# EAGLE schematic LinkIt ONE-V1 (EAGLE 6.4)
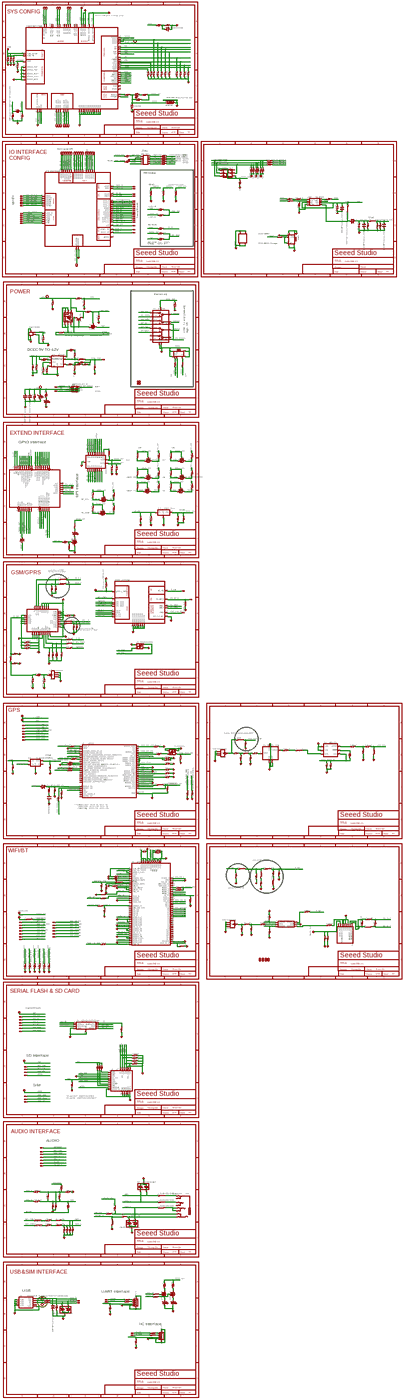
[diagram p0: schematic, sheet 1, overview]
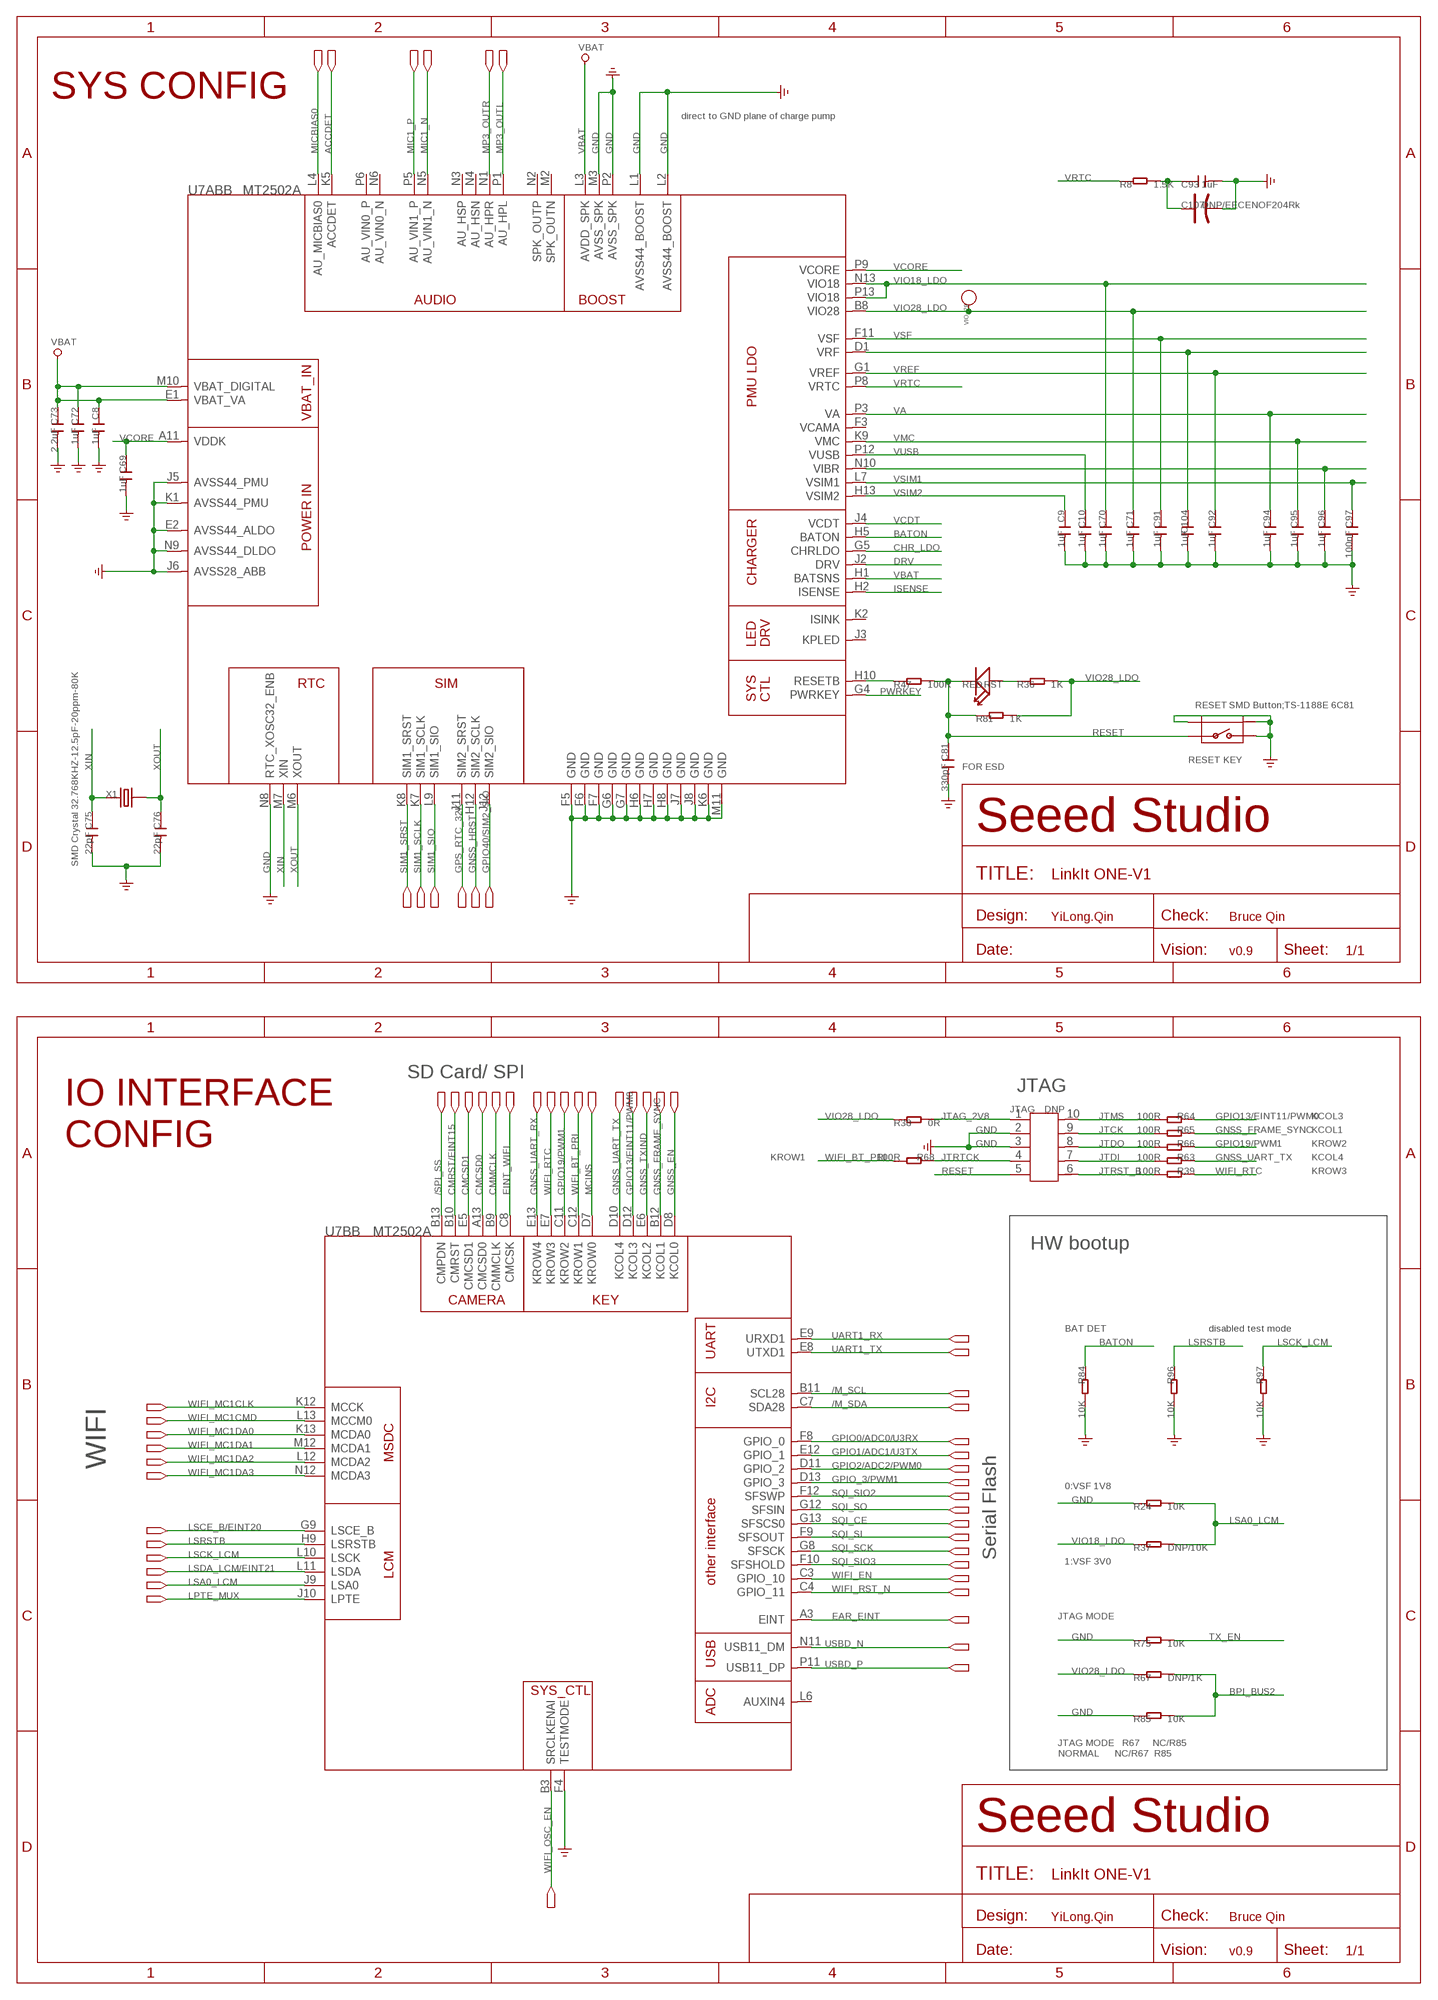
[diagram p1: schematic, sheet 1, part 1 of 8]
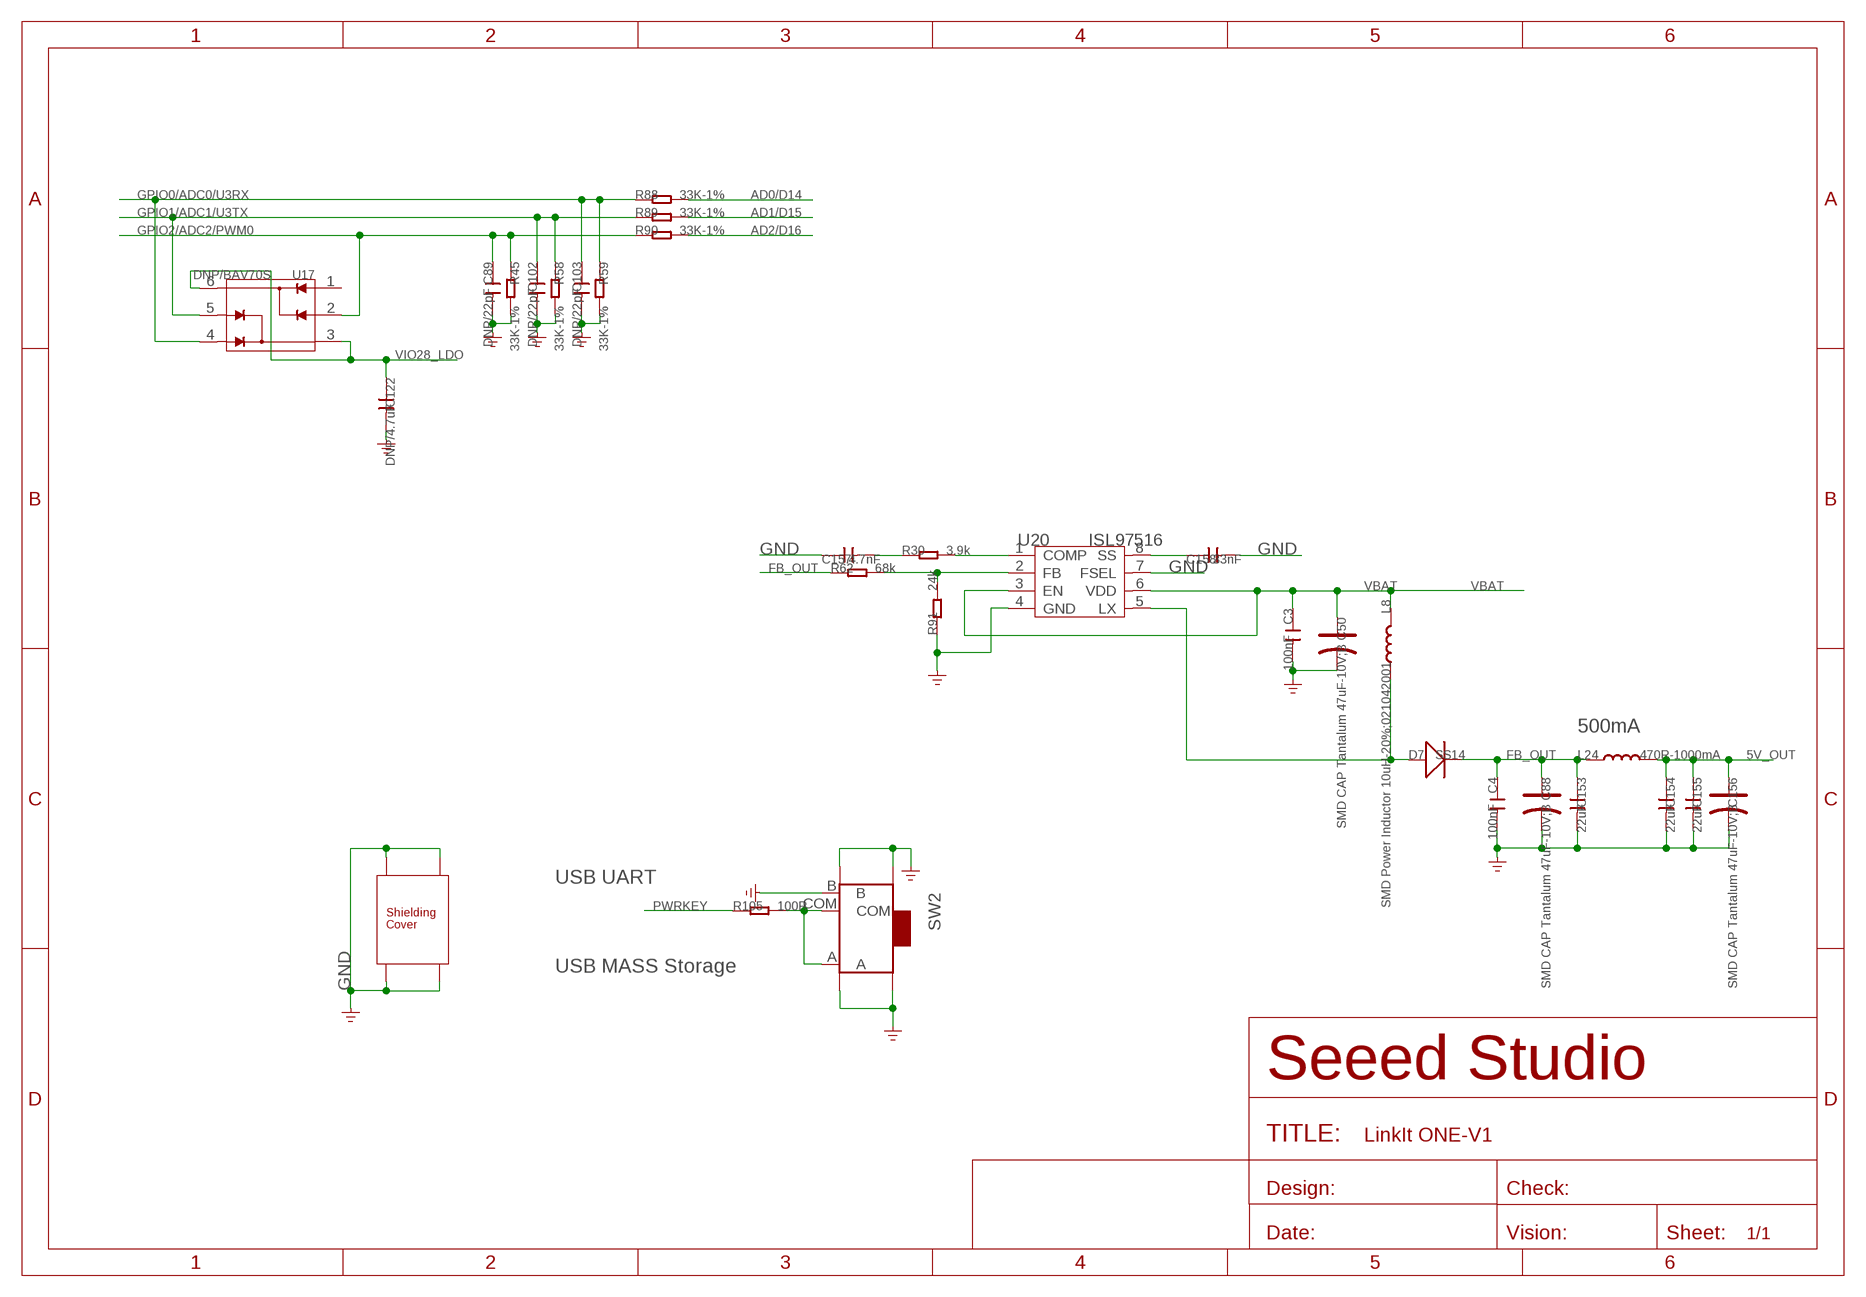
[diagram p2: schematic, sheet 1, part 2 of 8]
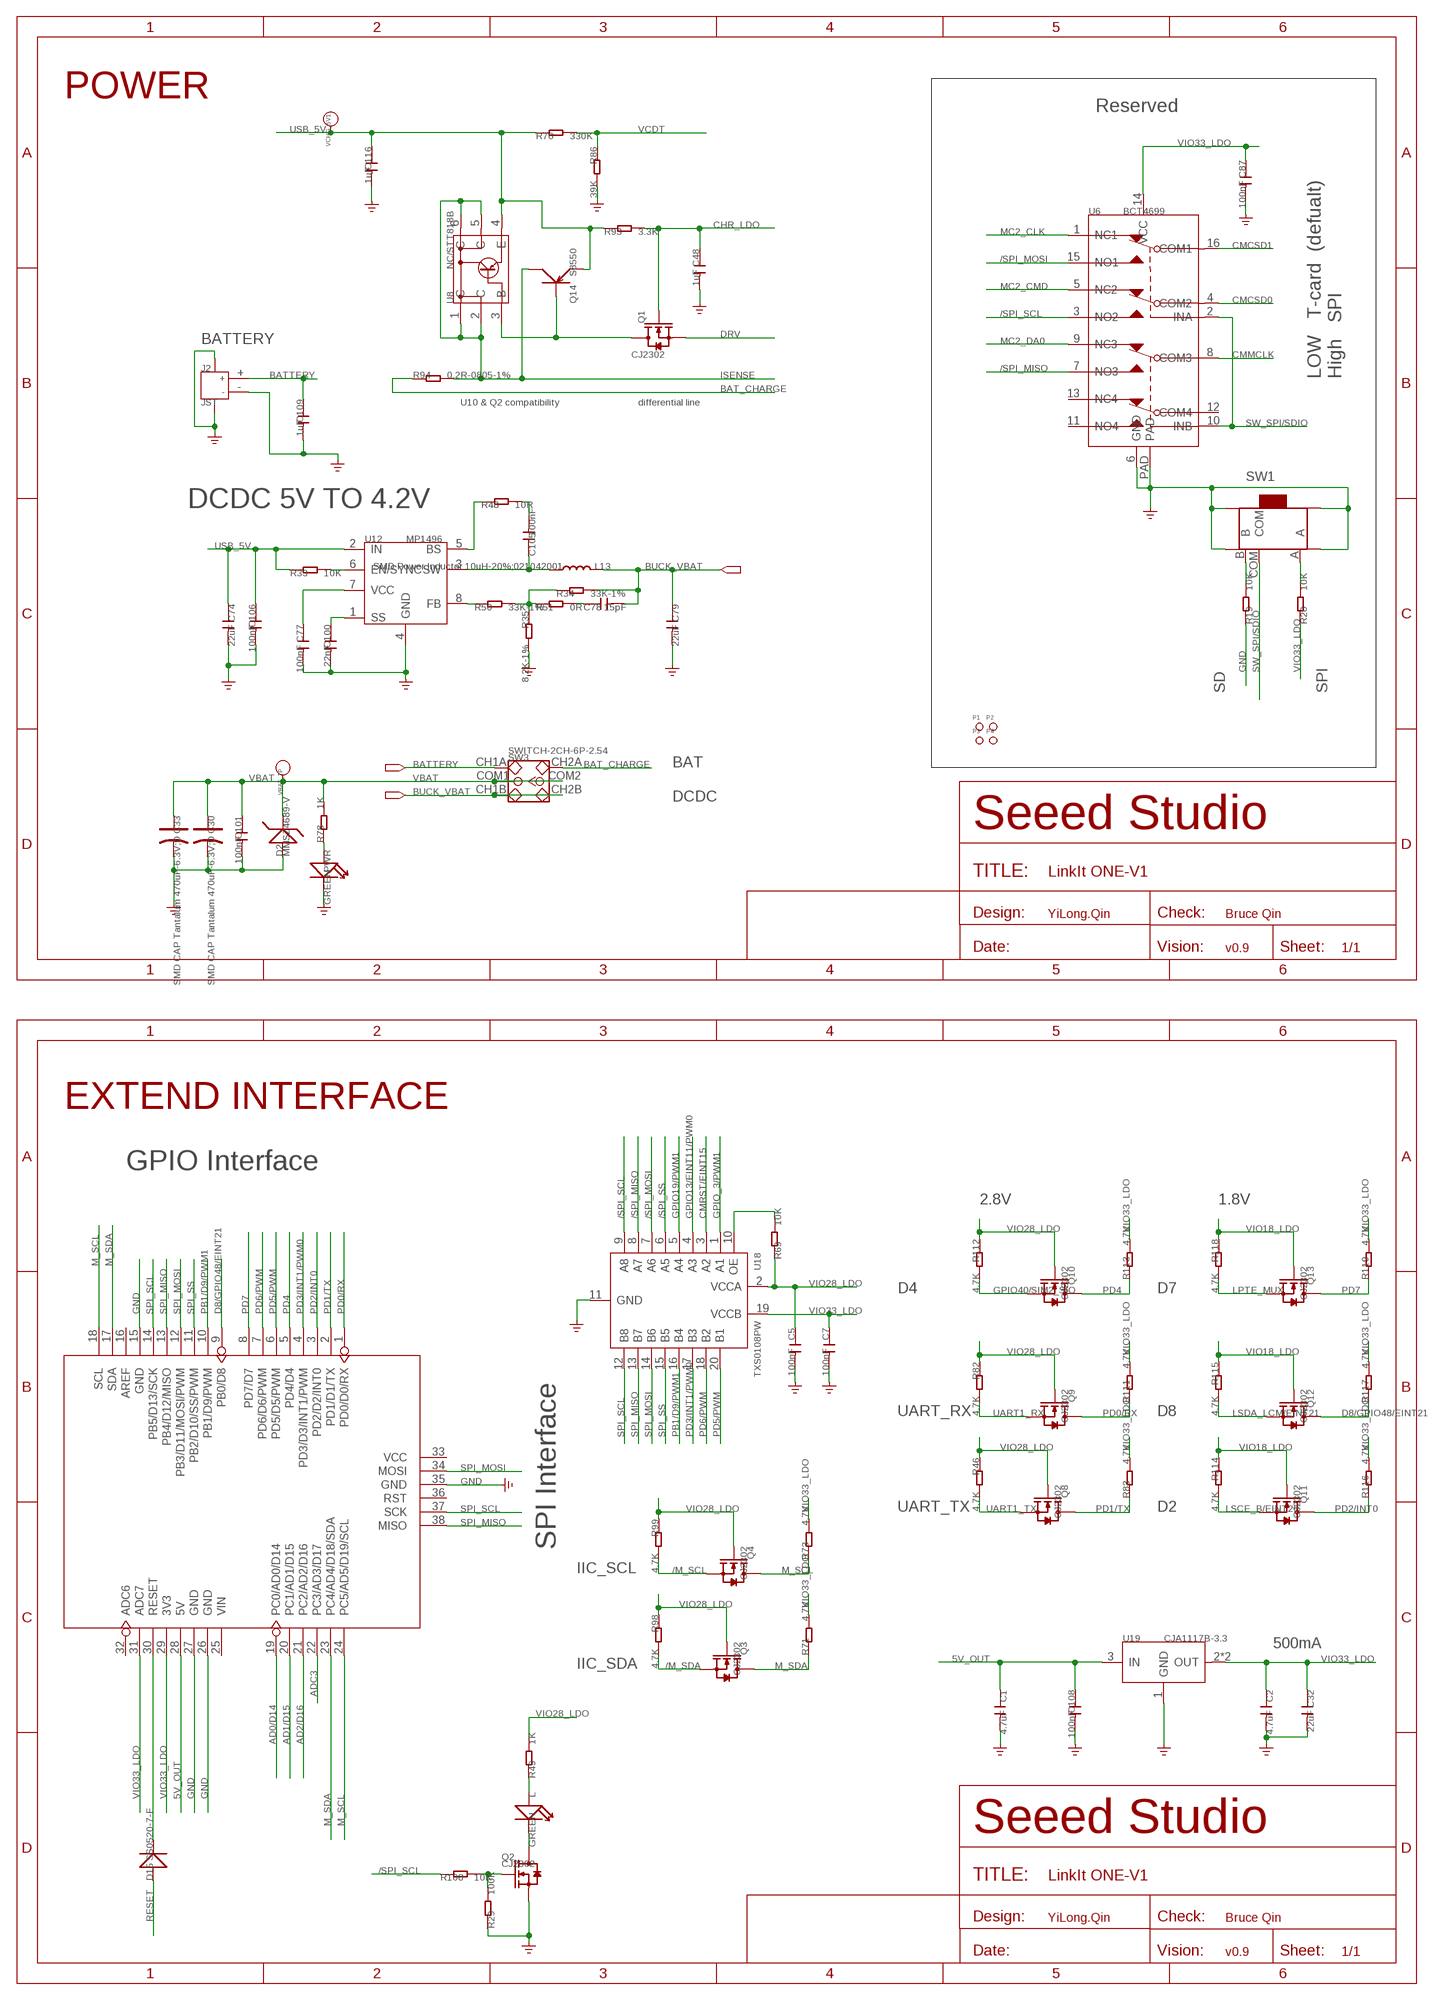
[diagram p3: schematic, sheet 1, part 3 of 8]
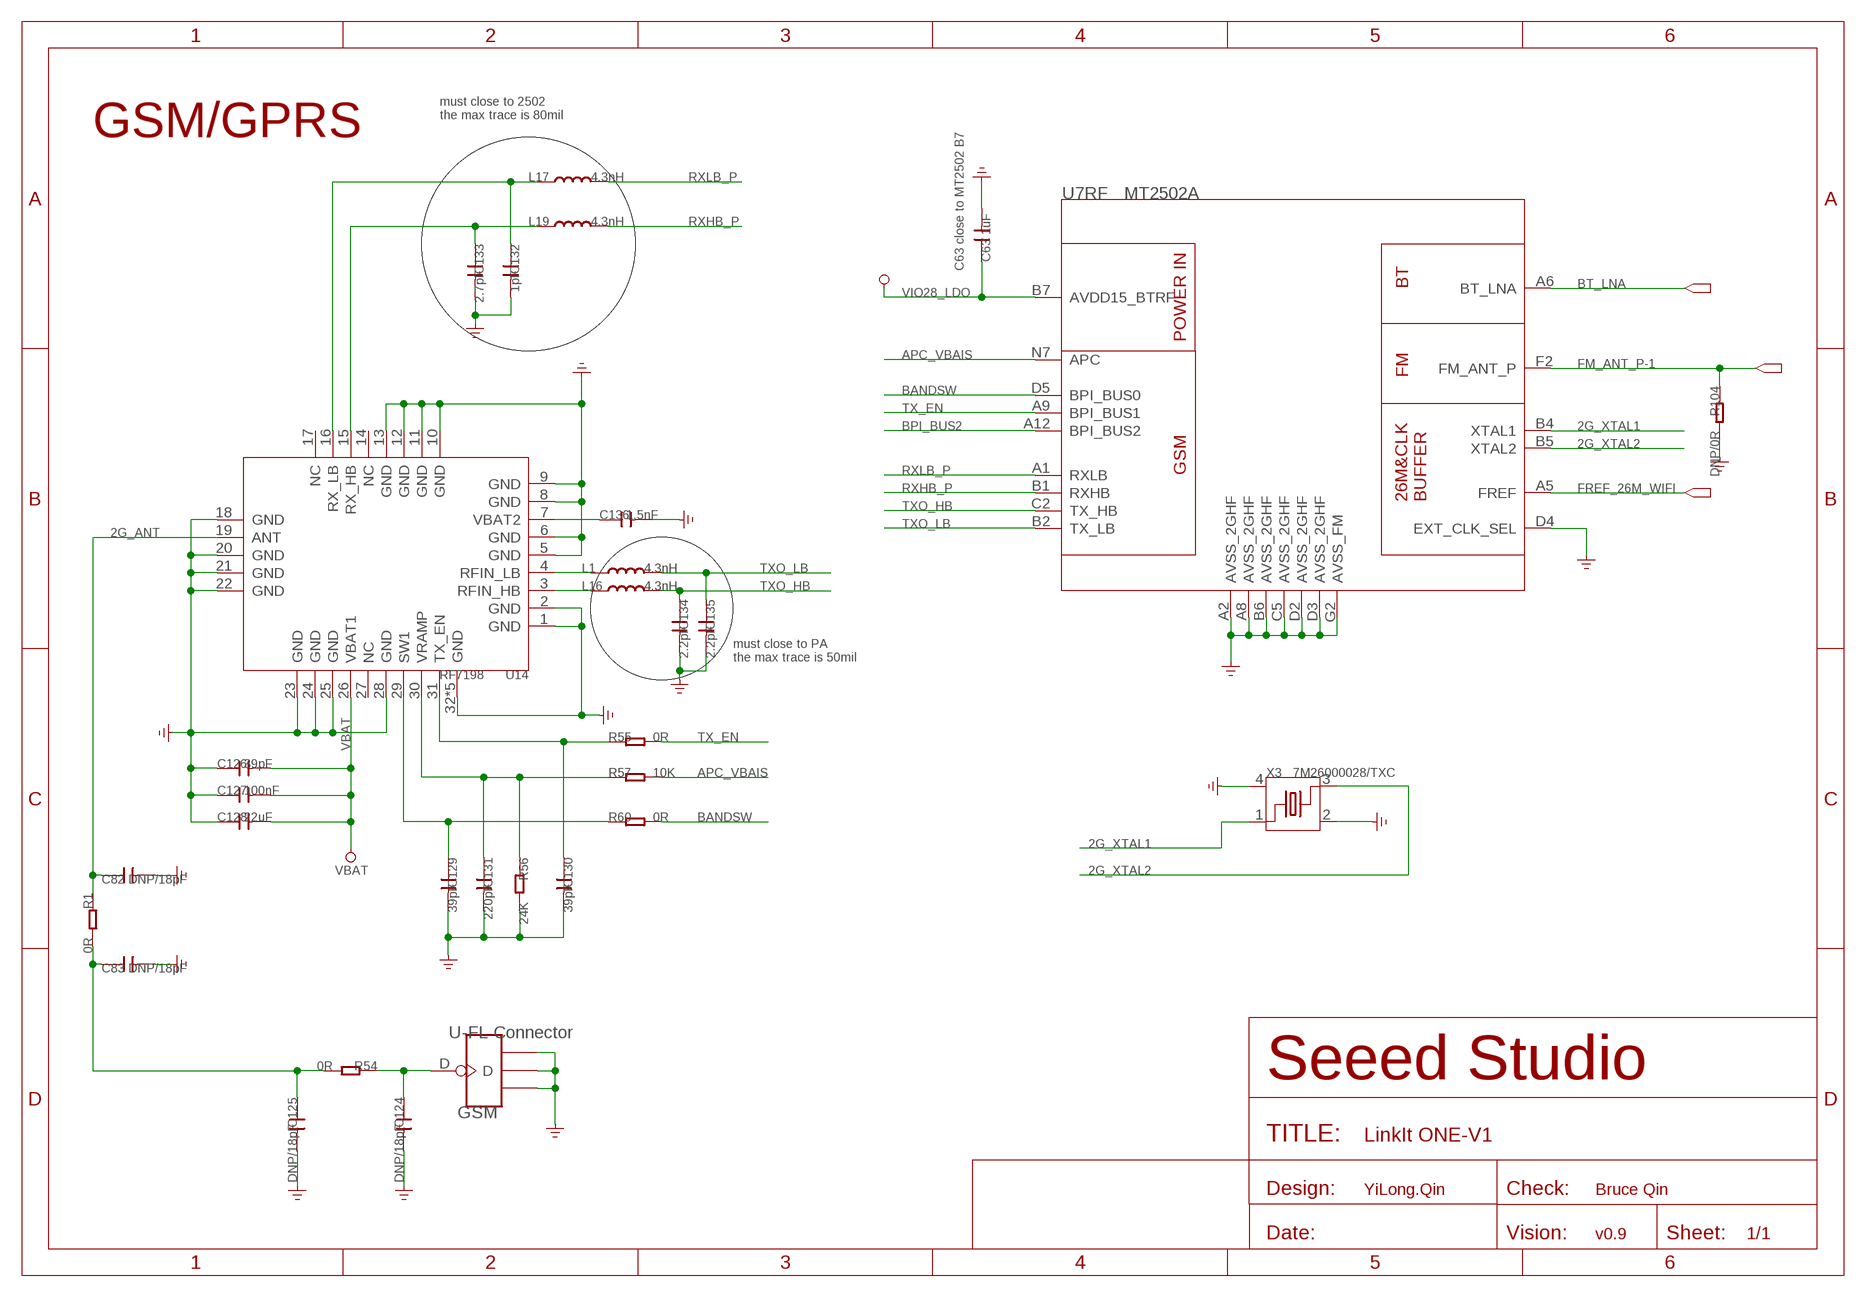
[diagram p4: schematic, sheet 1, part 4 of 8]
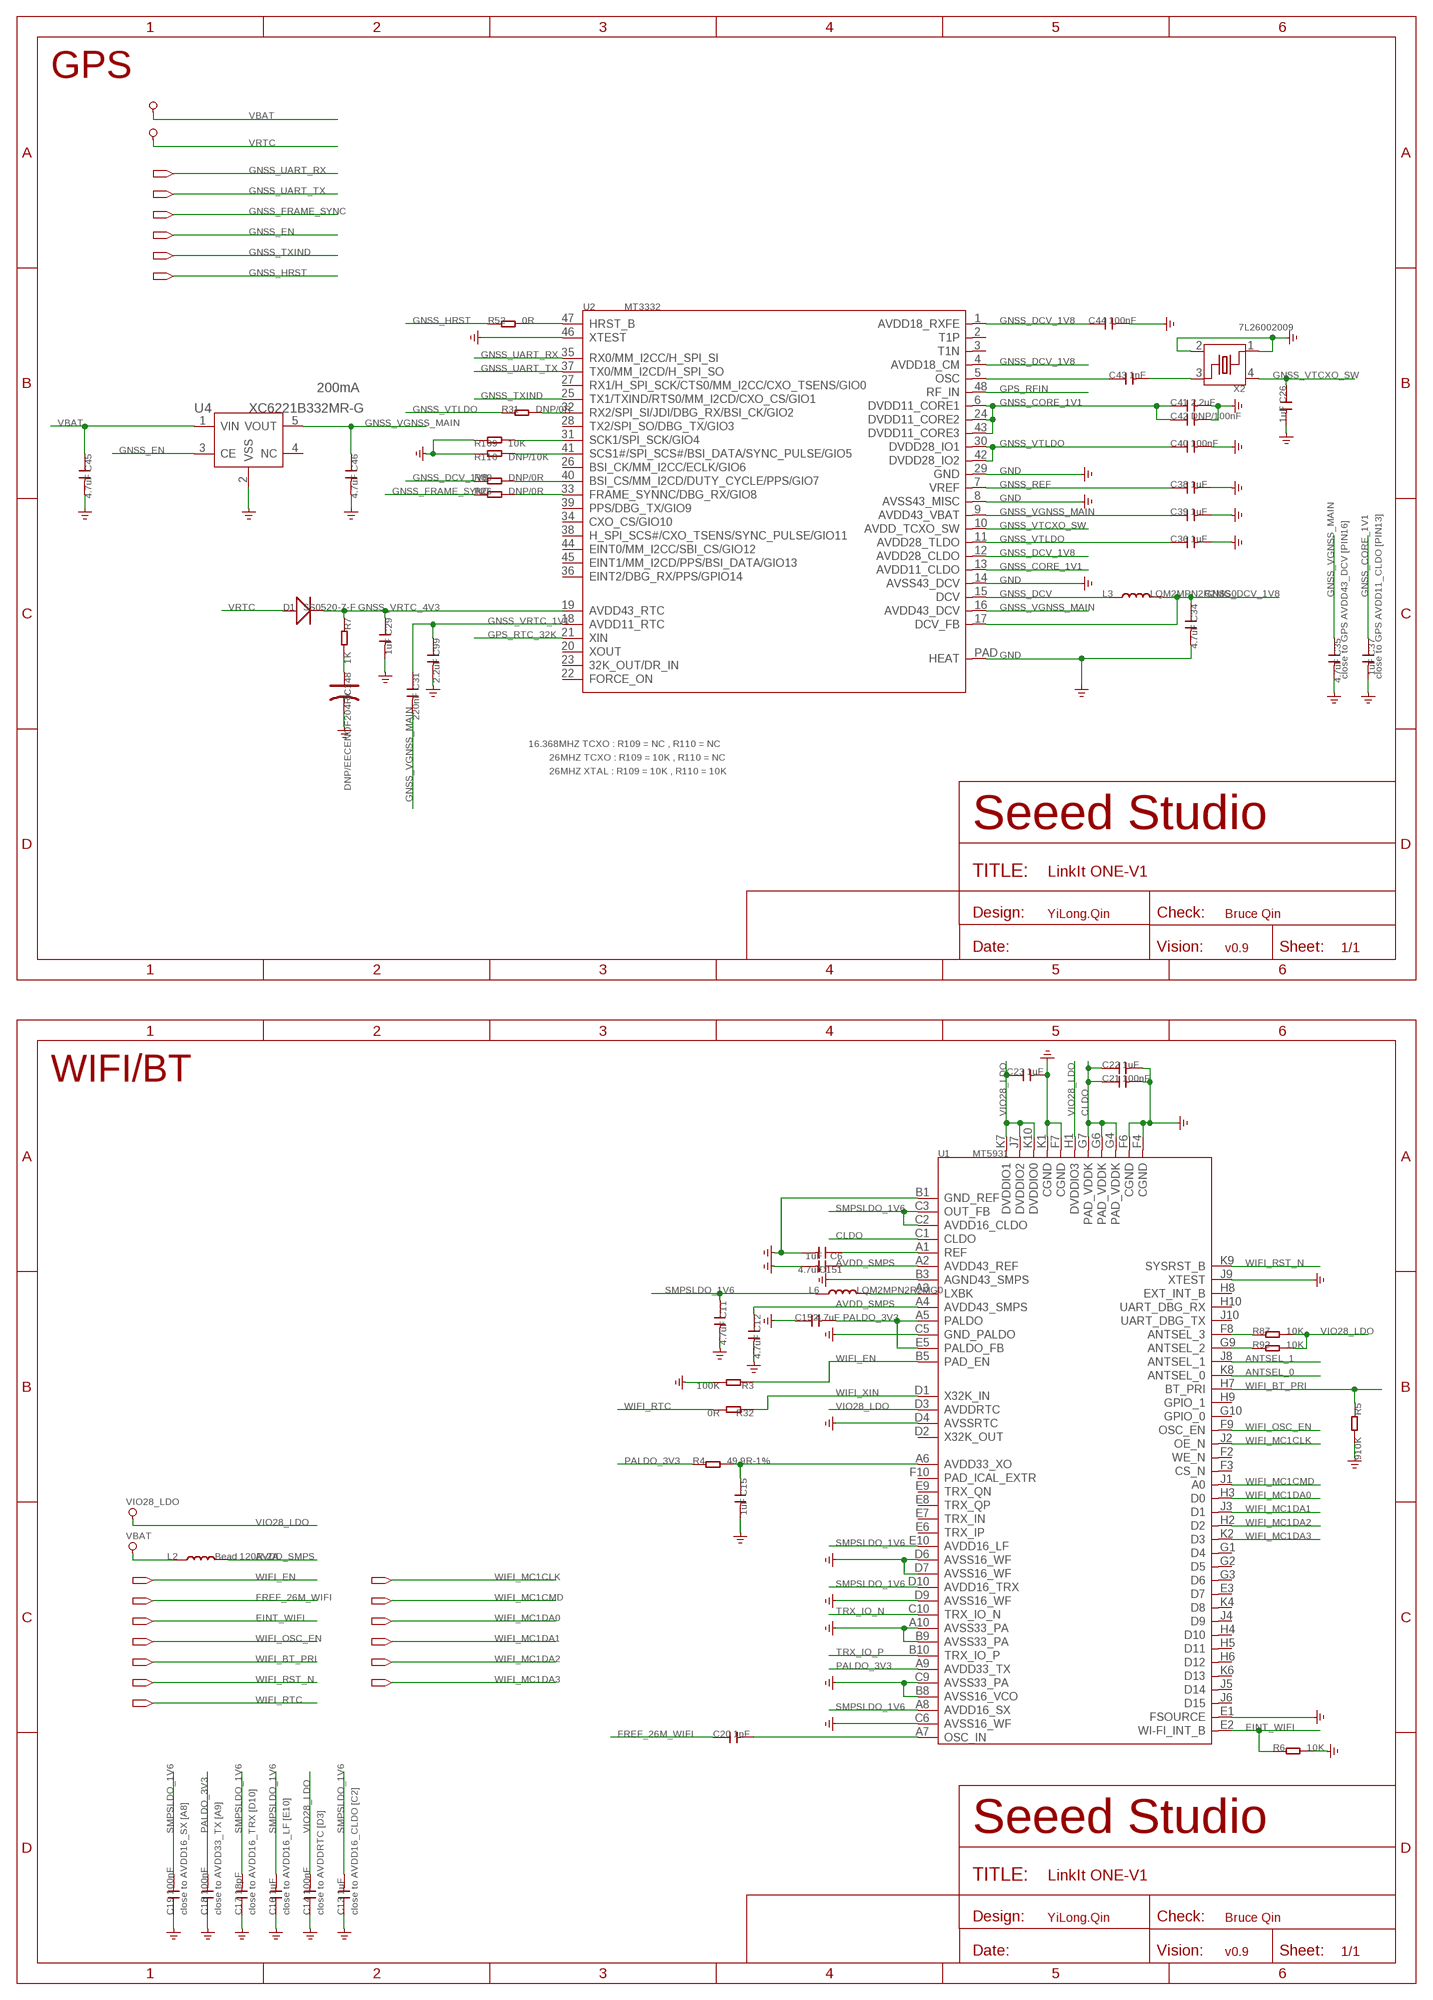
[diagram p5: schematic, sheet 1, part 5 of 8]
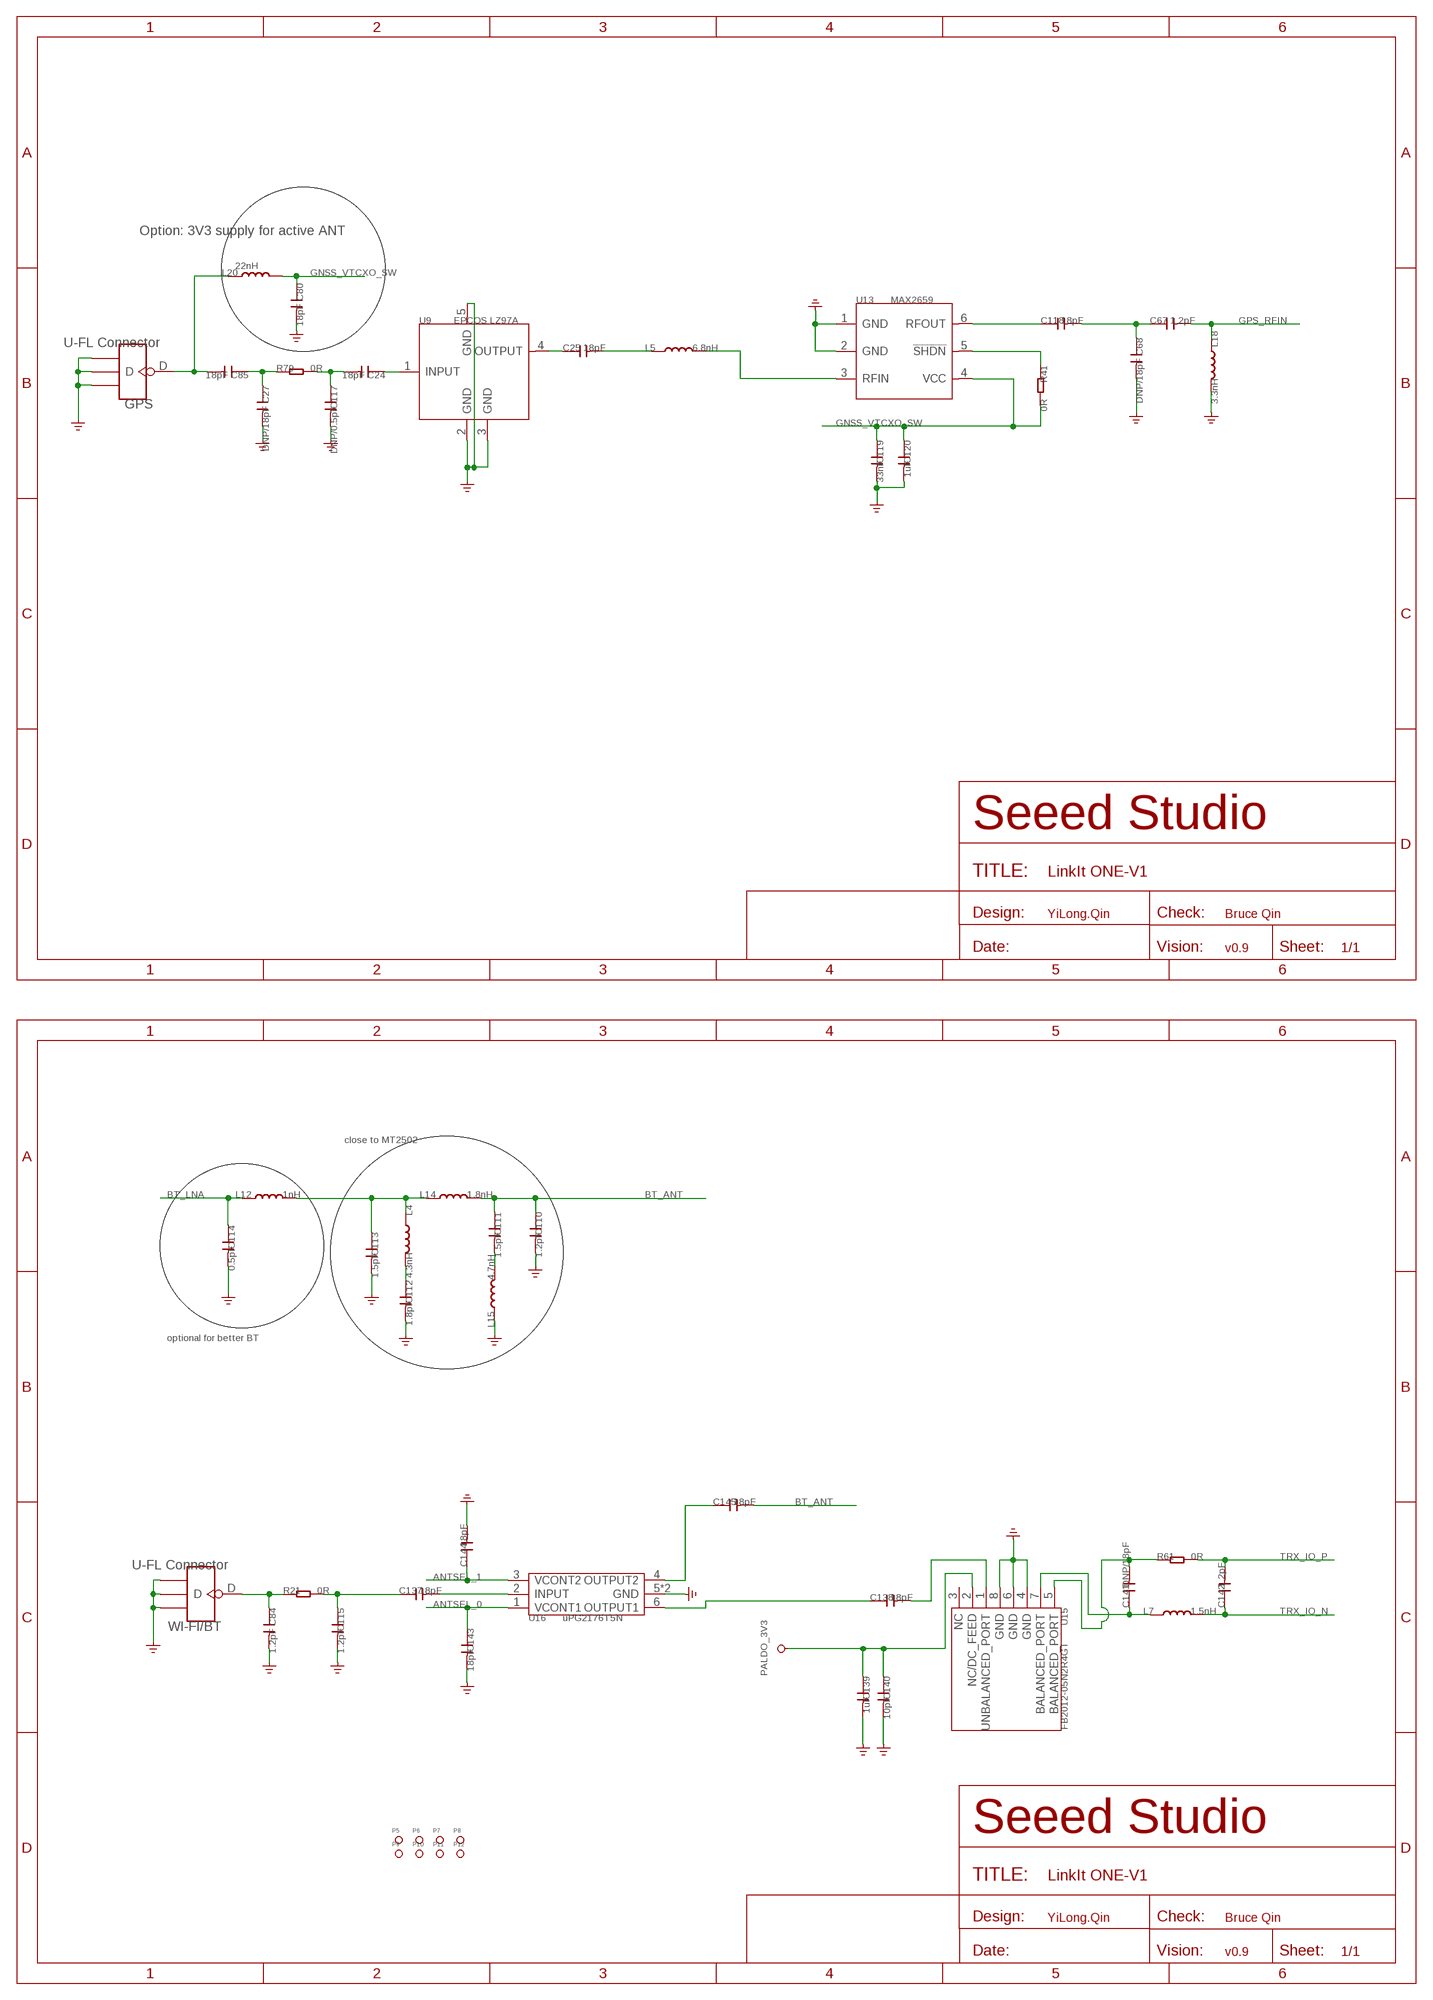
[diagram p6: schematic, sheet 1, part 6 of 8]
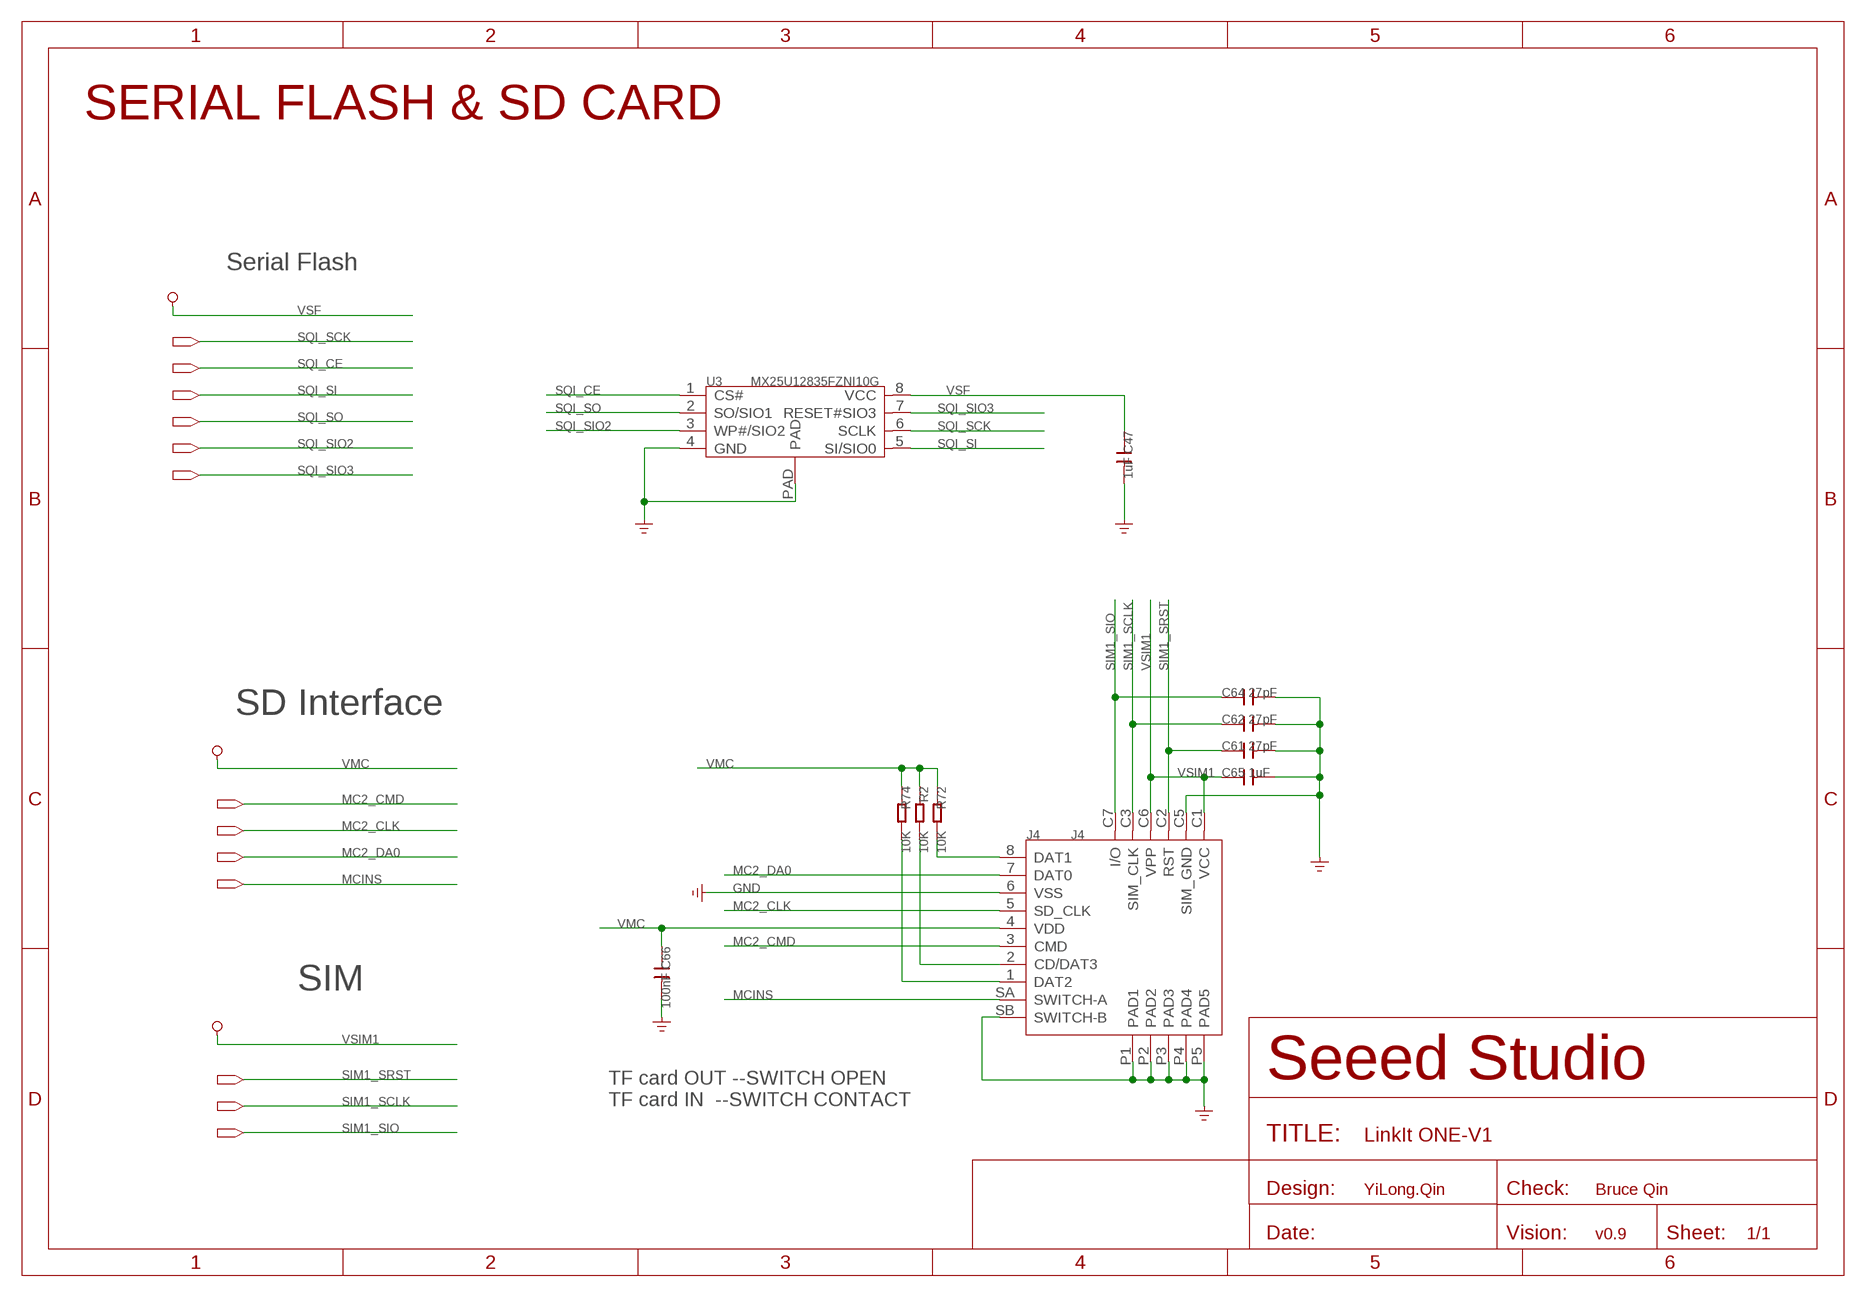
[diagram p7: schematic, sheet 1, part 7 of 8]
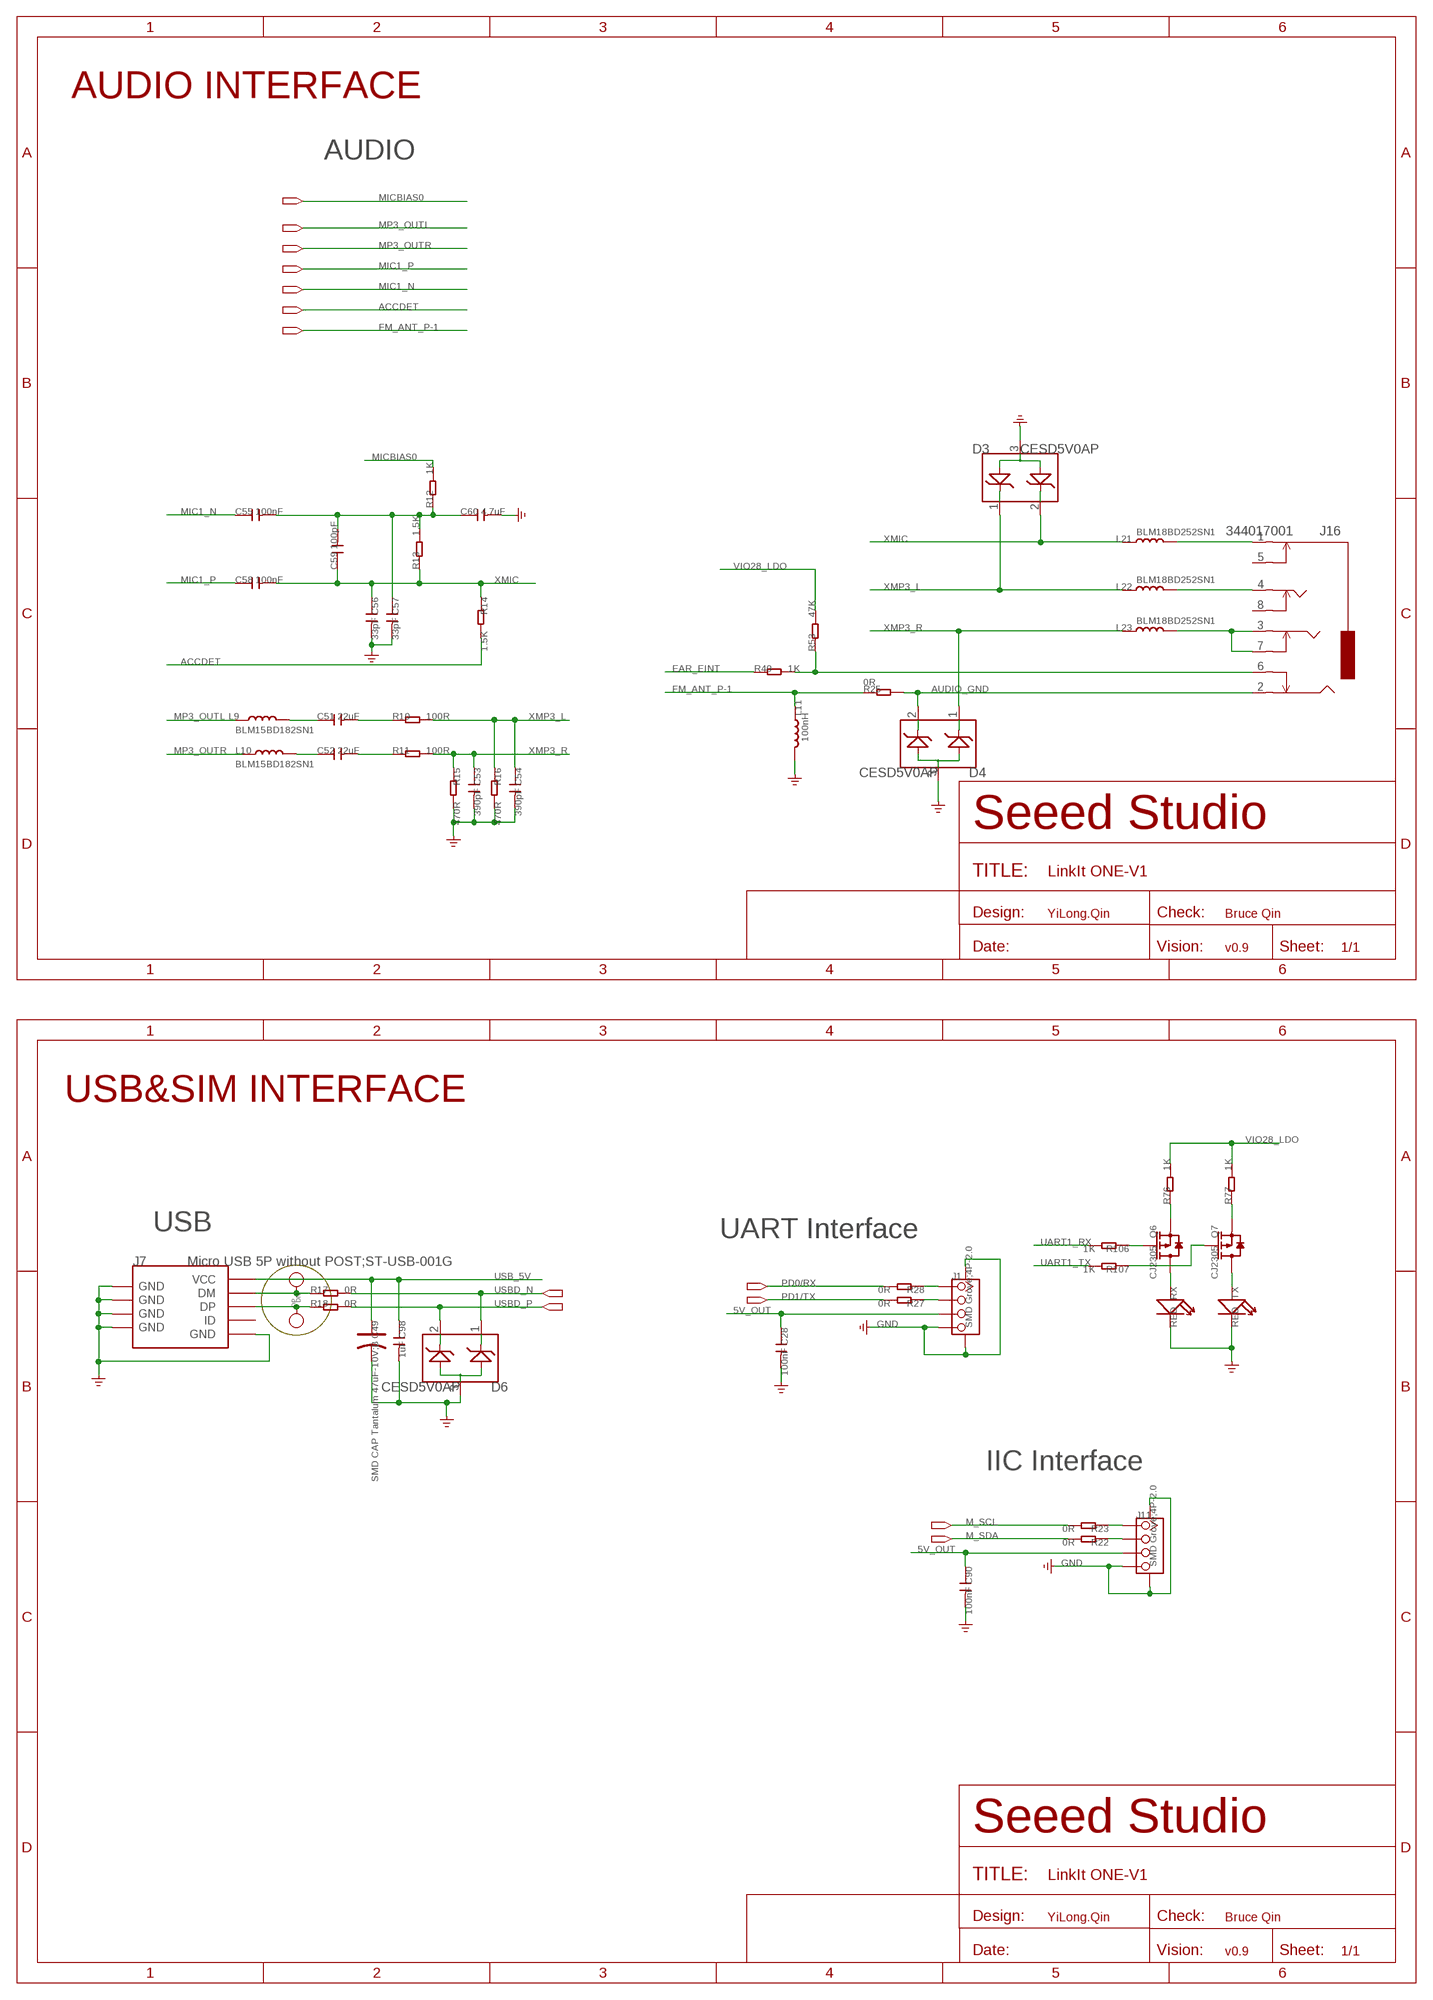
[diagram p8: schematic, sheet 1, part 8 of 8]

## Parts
C1  4.7uF  C-0805  [C0805]
C2  4.7uF  C-0805  [C0805]
C3  100nF  C-0402  [C0402]
C4  100nF  C-0402  [C0402]
C5  100nF  C-0402  [C0402]
C6  1uF  C-0402  [C0402]
C7  100nF  C-0402  [C0402]
C8  1uF  C-0402  [C0402]
C9  1uF  C-0402  [C0402]
C10  1uF  C-0402  [C0402]
C11  4.7uF  C-0805  [C0805]
C12  4.7uF  C-0805  [C0805]
C13  1uF  C-0402  [C0402]
C14  100nF  C-0402  [C0402]
C15  1uF  C-0402  [C0402]
C16  1uF  C-0402  [C0402]
C17  18pF  C-0402  [C0402]
C18  100nF  C-0402  [C0402]
C19  100nF  C-0402  [C0402]
C20  1nF  C-0402  [C0402]
C21  100nF  C-0402  [C0402]
C22  1uF  C-0402  [C0402]
C23  1uF  C-0402  [C0402]
C24  18pF  C-0402  [C0402]
C25  18pF  C-0402  [C0402]
C26  1uF  C-0402  [C0402]
C27  DNP/18pF  C-0402  [C0402]
C28  100nF  C-0402  [C0402]
C29  1uF  C-0402  [C0402]
C30  SMD CAP Tantalum 470uF-6.3V;D  CAP-AVX-D  [AVX-D]
C31  220nF  C-0402  [C0402]
C32  22uF  C-0805  [C0805]
C33  SMD CAP Tantalum 470uF-6.3V;D  CAP-AVX-D  [AVX-D]
C34  4.7uF  C-0805  [C0805]
C35  4.7uF  C-0805  [C0805]
C36  1uF  C-0402  [C0402]
C37  1uF  C-0402  [C0402]
C38  1uF  C-0402  [C0402]
C39  1uF  C-0402  [C0402]
C40  100nF  C-0402  [C0402]
C41  2.2uF  C-0603  [C0603]
C42  DNP/100nF  C-0402  [C0402]
C43  1nF  C-0402  [C0402]
C44  100nF  C-0402  [C0402]
C45  4.7uF  C-0805  [C0805]
C46  4.7uF  C-0805  [C0805]
C47  1uF  C-0402  [C0402]
C48  1uF  C-0402  [C0402]
C49  SMD CAP Tantalum 47uF-10V;B  CAP-AVX-B  [AVX-B]
C50  SMD CAP Tantalum 47uF-10V;B  CAP-AVX-B  [AVX-B]
C51  22uF  C-0805  [C0805]
C52  22uF  C-0805  [C0805]
C53  390pF  C-0402  [C0402]
C54  390pF  C-0402  [C0402]
C55  100nF  C-0402  [C0402]
C56  33pF  C-0402  [C0402]
C57  33pF  C-0402  [C0402]
C58  100nF  C-0402  [C0402]
C59  100pF  C-0402  [C0402]
C60  4.7uF  C-0805  [C0805]
C61  27pF  C-0402  [C0402]
C62  27pF  C-0402  [C0402]
C63  1uF  C-0402  [C0402]
C64  27pF  C-0402  [C0402]
C65  1uF  C-0402  [C0402]
C66  100nF  C-0402  [C0402]
C67  1.2pF  C-0402  [C0402]
C68  DNP/18pF  C-0402  [C0402]
C69  1uF  C-0402  [C0402]
C70  1uF  C-0402  [C0402]
C71  1uF  C-0402  [C0402]
C72  1uF  C-0402  [C0402]
C73  2.2uF  C-0603  [C0603]
C74  22uF  C-0805  [C0805]
C75  22pF  C-0402  [C0402]
C76  22pF  C-0402  [C0402]
C77  100nF  C-0402  [C0402]
C78  15pF  C-0402  [C0402]
C79  22uF  C-0805  [C0805]
C80  18pF  C-0402  [C0402]
C81  330pF  C-0402  [C0402]
C82  DNP/18pF  C-0402  [C0402]
C83  DNP/18pF  C-0402  [C0402]
C84  1.2pF  C-0402  [C0402]
C85  18pF  C-0402  [C0402]
C87  100nF  C-0402  [C0402]
C88  SMD CAP Tantalum 47uF-10V;B  CAP-AVX-B  [AVX-B]
C89  DNP/22pF  C-0402  [C0402]
C90  100nF  C-0402  [C0402]
C91  1uF  C-0402  [C0402]
C92  1uF  C-0402  [C0402]
C93  1uF  C-0402  [C0402]
C94  1uF  C-0402  [C0402]
C95  1uF  C-0402  [C0402]
C96  1uF  C-0402  [C0402]
C97  100nF  C-0402  [C0402]
C98  1uF  C-0402  [C0402]
C99  2.2uF  C-0603  [C0603]
C100  22nF  C-0402  [C0402]
C101  100nF  C-0402  [C0402]
C102  DNP/22pF  C-0402  [C0402]
C103  DNP/22pF  C-0402  [C0402]
C104  1uF  C-0402  [C0402]
C105  100nF  C-0402  [C0402]
C106  100nF  C-0402  [C0402]
C107  DNP/EECENOF204Rk  C-ELECTRIC-DOUBLE-LAYER-CAPACITOR  [2P-D6.8MMX1.8MMH]
C108  100nF  C-0402  [C0402]
C109  1uF  C-0402  [C0402]
C110  1.2pF  C-0402  [C0402]
C111  1.5pF  C-0402  [C0402]
C112  1.8pF  C-0402  [C0402]
C113  1.5pF  C-0402  [C0402]
C114  0.5pF  C-0402  [C0402]
C115  1.2pF  C-0402  [C0402]
C116  1uF  C-0402  [C0402]
C117  DNP/0.5pF  C-0402  [C0402]
C118  18pF  C-0402  [C0402]
C119  33nF  C-0402  [C0402]
C120  1uF  C-0402  [C0402]
C122  DNP/4.7uF  C-0805  [C0805]
C124  DNP/18pF  C-0402  [C0402]
C125  DNP/18pF  C-0402  [C0402]
C126  39pF  C-0402  [C0402]
C127  100nF  C-0402  [C0402]
C128  22uF  C-0805  [C0805]
C129  39pF  C-0402  [C0402]
C130  39pF  C-0402  [C0402]
C131  220pF  C-0402  [C0402]
C132  1pF  C-0402  [C0402]
C133  2.7pF  C-0402  [C0402]
C134  2.2pF  C-0402  [C0402]
C135  2.2pF  C-0402  [C0402]
C136  1.5nF  C-0402  [C0402]
C137  18pF  C-0402  [C0402]
C138  18pF  C-0402  [C0402]
C139  1uF  C-0402  [C0402]
C140  10pF  C-0402  [C0402]
C141  DNP/18pF  C-0402  [C0402]
C142  1.2pF  C-0402  [C0402]
C143  18pF  C-0402  [C0402]
C144  18pF  C-0402  [C0402]
C145  18pF  C-0402  [C0402]
C148  DNP/EECENOF204Rk  C-ELECTRIC-DOUBLE-LAYER-CAPACITOR  [2P-D6.8MMX1.8MMH]
C151  4.7uF  C-0805  [C0805]
C152  4.7uF  C-0805  [C0805]
C153  22uF  C-0805  [C0805]
C154  22uF  C-0805  [C0805]
C155  22uF  C-0805  [C0805]
C156  SMD CAP Tantalum 47uF-10V;B  CAP-AVX-B  [AVX-B]
C157  4.7nF  C-0402  [C0402]
C158  33nF  C-0402  [C0402]
D1  SS0520-7-F  D'1206'  [SOD123]
D2  MMSZ4689-V  D-VOL'MMSZ4681'  [SOD123-2.7X1.6]
D3  CESD5V0AP  D-ESD-3P  [SOT23]
D4  CESD5V0AP  D-ESD-3P  [SOT23]
D6  CESD5V0AP  D-ESD-3P  [SOT23]
D7  SS14  D'DO-214AC'  [D2010]
D15  SS0520-7-F  D'1206'  [SOD123]
DN  USB_DP  PAD-TEST-POINT'4545'  [TP_4545]
DP  USB_DN  PAD-TEST-POINT'4545'  [TP_4545]
GPS  U-FL Connector  ANTENNA-U-FL  [4P-U-FL]
GSM  U-FL Connector  ANTENNA-U-FL  [4P-U-FL]
J1  SMD Grove;4P-2.0  TWIG-4P-2.0-SMD-FEMALE-REINFORCE'DD'  [4P-SMD-2.0]
J2  JST  JACK-JST-2P-SMD-PW'2.0'  [JST-SMD-2.0-90D]
J4  TF+SIM-VSHO-21-3301  HOLDER-SD/SIM-CONNECTER'VSHO-21-3301'  [16P-L17.4MM*W16.5MM*H2.7MM]
J7  Micro USB 5P without POST;ST-USB-001G  USB-MINIUSB-5P-MICRO  [MICRO-USB]
J11  SMD Grove;4P-2.0  TWIG-4P-2.0-SMD-FEMALE-REINFORCE'DD'  [4P-SMD-2.0]
J16  344017001  AUDIO-8P-SMD'PJ-3536-L6S'  [8P-3.5-SMD]
JTAG  DNP  HEADER-2X5P-2.0  [2*5P-2.0-TESTPOINT]
L  GREEN  LED'0603'  [LED-0603]
L1  4.3nH  L'0402'  [L0402]
L2  Bead 120R-2A  L'0603'  [L0603]
L3  LQM2MPN2R2MG0  L'0806'  [0806]
L4  4.3nH  L'0402'  [L0402]
L5  6.8nH  L'0402'  [L0402]
L6  LQM2MPN2R2MG0  L'0806'  [0806]
L7  1.5nH  L'0402'  [L0402]
L8  SMD Power Inductor 10uH-20%;021042001  L'0630'  [L0630]
L9  BLM15BD182SN1  L'0402'  [L0402]
L10  BLM15BD182SN1  L'0402'  [L0402]
L11  100nH  L'0603'  [L0603]
L12  1nH  L'0402'  [L0402]
L13  SMD Power Inductor 10uH-20%;021042001  L'0630'  [L0630]
L14  1.8nH  L'0402'  [L0402]
L15  4.7nH  L'0402'  [L0402]
L16  4.3nH  L'0402'  [L0402]
L17  4.3nH  L'0402'  [L0402]
L18  3.3nH  L'0402'  [L0402]
L19  4.3nH  L'0402'  [L0402]
L20  22nH  L'0603'  [L0603]
L21  BLM18BD252SN1  L'0603'  [L0603]
L22  BLM18BD252SN1  L'0603'  [L0603]
L23  BLM18BD252SN1  L'0603'  [L0603]
L24  470R-1000mA  L'0805'  [L0805]
P1  PAD-MARK'ANNULAR'  [ROUND-MARK-1.0]
P2  PAD-MARK'ANNULAR'  [ROUND-MARK-1.0]
P3  PAD-MARK'ANNULAR'  [ROUND-MARK-1.0]
P4  PAD-MARK'ANNULAR'  [ROUND-MARK-1.0]
P5  PAD-MARK'ANNULAR'  [ROUND-MARK-1.0]
P6  PAD-MARK'ANNULAR'  [ROUND-MARK-1.0]
P7  PAD-MARK'ANNULAR'  [ROUND-MARK-1.0]
P8  PAD-MARK'ANNULAR'  [ROUND-MARK-1.0]
P9  PAD-MARK'ANNULAR'  [ROUND-MARK-1.0]
P10  PAD-MARK'ANNULAR'  [ROUND-MARK-1.0]
P11  PAD-MARK'ANNULAR'  [ROUND-MARK-1.0]
P12  PAD-MARK'ANNULAR'  [ROUND-MARK-1.0]
PWR  GREEN  LED'0603'  [LED-0603]
Q1  CJ2302  MOSFET-N'SOT23'  [SOT23]
Q2  CJ2302  MOSFET-N'SOT23'  [SOT23]
Q3  CJ2302  MOSFET-N'SOT23'  [SOT23]
Q4  CJ2302  MOSFET-N'SOT23'  [SOT23]
Q6  CJ2305  MOSFET-P'SI2323CDS/SI2305DS<BR>'  [SOT23]
Q7  CJ2305  MOSFET-P'SI2323CDS/SI2305DS<BR>'  [SOT23]
Q8  CJ2302  MOSFET-N'SOT23'  [SOT23]
Q9  CJ2302  MOSFET-N'SOT23'  [SOT23]
Q10  CJ2302  MOSFET-N'SOT23'  [SOT23]
Q11  CJ2302  MOSFET-N'SOT23'  [SOT23]
Q12  CJ2302  MOSFET-N'SOT23'  [SOT23]
Q13  CJ2302  MOSFET-N'SOT23'  [SOT23]
Q14  S8550  TRANSISTOR-PNP-SOT23  [SOT23]
R1  0R  R-0402  [R0402]
R2  10K  R-0402  [R0402]
R3  100K  R-0402  [R0402]
R4  49.9R-1%  R-0402  [R0402]
R5  910K  R-0402  [R0402]
R6  10K  R-0402  [R0402]
R7  1K  R-0402  [R0402]
R8  1.5K  R-0402  [R0402]
R10  100R  R-0402  [R0402]
R11  100R  R-0402  [R0402]
R12  1K  R-0402  [R0402]
R13  1.5K  R-0402  [R0402]
R14  1.5K  R-0402  [R0402]
R15  470R  R-0402  [R0402]
R16  470R  R-0402  [R0402]
R17  0R  R-0402  [R0402]
R18  0R  R-0402  [R0402]
R19  10K  R-0402  [R0402]
R20  10K  R-0402  [R0402]
R21  0R  R-0402  [R0402]
R22  0R  R-0402  [R0402]
R23  0R  R-0402  [R0402]
R24  10K  R-0402  [R0402]
R25  0R  R-0402  [R0402]
R26  DNP/0R  R-0402  [R0402]
R27  0R  R-0402  [R0402]
R28  0R  R-0402  [R0402]
R29  100K  R-0402  [R0402]
R30  3.9k  R-0402  [R0402]
R31  DNP/0R  R-0402  [R0402]
R32  0R  R-0402  [R0402]
R33  10K  R-0402  [R0402]
R34  33K-1%  R-0402  [R0402]
R35  8.2K-1%  R-0402  [R0402]
R36  1K  R-0402  [R0402]
R37  DNP/10K  R-0402  [R0402]
R38  0R  R-0402  [R0402]
R39  100R  R-0402  [R0402]
R40  1K  R-0402  [R0402]
R41  0R  R-0402  [R0402]
R45  33K-1%  R-0402  [R0402]
R46  4.7K  R-0402  [R0402]
R47  100R  R-0402  [R0402]
R48  10R  R-0402  [R0402]
R49  1K  R-0402  [R0402]
R50  33K-1%  R-0402  [R0402]
R51  0R  R-0402  [R0402]
R52  0R  R-0402  [R0402]
R53  47K  R-0402  [R0402]
R54  0R  R-0402  [R0402]
R55  0R  R-0402  [R0402]
R56  24K  R-0402  [R0402]
R57  10K  R-0402  [R0402]
R58  33K-1%  R-0402  [R0402]
R59  33K-1%  R-0402  [R0402]
R60  0R  R-0402  [R0402]
R61  0R  R-0402  [R0402]
R62  68k  R-0402  [R0402]
R63  100R  R-0402  [R0402]
R64  100R  R-0402  [R0402]
R65  100R  R-0402  [R0402]
R66  100R  R-0402  [R0402]
R67  DNP/1K  R-0402  [R0402]
R68  100R  R-0402  [R0402]
R69  10K  R-0402  [R0402]
R70  330K  R-0402  [R0402]
R71  4.7K  R-0402  [R0402]
R72  10K  R-0402  [R0402]
R73  4.7K  R-0402  [R0402]
R74  10K  R-0402  [R0402]
R75  10K  R-0402  [R0402]
R76  1K  R-0402  [R0402]
R77  1K  R-0402  [R0402]
R78  1K  R-0402  [R0402]
R79  0R  R-0402  [R0402]
R80  DNP/0R  R-0402  [R0402]
R81  1K  R-0402  [R0402]
R82  4.7K  R-0402  [R0402]
R83  4.7K  R-0402  [R0402]
R84  10K  R-0402  [R0402]
R85  10K  R-0402  [R0402]
R86  39K  R-0402  [R0402]
R87  10K  R-0402  [R0402]
R88  33K-1%  R-0402  [R0402]
R89  33K-1%  R-0402  [R0402]
R90  33K-1%  R-0402  [R0402]
R91  24k  R-0402  [R0402]
R92  10K  R-0402  [R0402]
R93  3.3K  R-0402  [R0402]
R94  0.2R-0805-1%  R-0805  [R0805]
R96  10K  R-0402  [R0402]
R97  10K  R-0402  [R0402]
R98  4.7K  R-0402  [R0402]
R99  4.7K  R-0402  [R0402]
R104  DNP/0R  R-0402  [R0402]
R105  100R  R-0402  [R0402]
R106  1K  R-0402  [R0402]
R107  1K  R-0402  [R0402]
R108  10K  R-0402  [R0402]
R109  10K  R-0402  [R0402]
R110  DNP/10K  R-0402  [R0402]
R111  4.7K  R-0402  [R0402]
R112  4.7K  R-0402  [R0402]
R113  4.7K  R-0402  [R0402]
R114  4.7K  R-0402  [R0402]
R115  4.7K  R-0402  [R0402]
R116  4.7K  R-0402  [R0402]
R117  4.7K  R-0402  [R0402]
R118  4.7K  R-0402  [R0402]
R119  4.7K  R-0402  [R0402]
RESET  SMD Button;TS-1188E 6C81  BUTTON-4P-REINFORCE'TS-1188E'  [4P-SMD-7X3.5X3.5H]
RST  RED  LED'0603'  [LED-0603]
RX  RED  LED'0603'  [LED-0603]
SW1  SWITCH-3P-SMD-6.6X2.8  [3P-SMD-2CH-6.6X2.8-REINFORCE]
SW2  SWITCH-3P-SMD-6.6X2.8  [3P-SMD-2CH-6.6X2.8-REINFORCE]
SW3  SWITCH-2CH-6P-2.54  SWITCH-2CH-6P  [6P-2CH-2.54-7.6X3.0]
TX  RED  LED'0603'  [LED-0603]
U1  MT5931  [TFBGA84]
U2  MT3332  [QFN48-6X6MM]
U3  MX25U12835FZNI10G  MX25U12835F  [WSON8-6X5X0.8H-W/HEAT]
U4  XC6221B332MR-G  XC6228  [SOT-25J]
U6  BCT4699  [TQFN16]
U7  MT2502A  [VFBGA143]
U8  NC/STT818B  STT818B  [SOT23-6L]
U9  EPCOS LZ97A  FILTER-FOR_GPS1500  [5P-SMD-1.4X1.1MM]
U10  SHIELDING-COVER  [SHIELD-SMD-44.5X53.5]
U11  PCB  ARDUINO-38P  [ARDUINO-38P]
U12  MP1496  MP1496DJ  [TSOT23-8]
U13  MAX2659  [6P-SMD-1.5X1.0X0.72H]
U14  RF7198  RF1798  [32P-SMD-RF1798-5.3MMX5.25MMX0.73H]
U15  FB2012-05N2R4GT  FILTER-FB2012  [8P-SMD-2X1.25X0.7H]
U16  uPG2176T5N  UPG2176T5N  [TSON6]
U17  DNP/BAV70S  BAV70S  [SOT363]
U18  TXS0108PW  TXS0108E  [TSSOP20]
U19  CJA1117B-3.3  LD1117'SOT89'  [SOT89]
U20  ISL97516  [MSOP8]
VBAT_TP  VBAT  PAD-TEST-POINT'4545'  [TP_4545]
VCHG_5V1  PAD-TEST-POINT'4545'  [TP_4545]
VIO_28  PAD-TEST-POINT'4545'  [TP_4545]
WI-FI/BT  U-FL Connector  ANTENNA-U-FL  [4P-U-FL]
X1  SMD Crystal 32.768KHZ-12.5pF-20ppm-80K  CRYSTAL'NX2012SA'  [2P-SMD-2.05X1.2]
X2  7L26002009  CRYSTAL'NX2520SA'  [2520]
X3  7M26000028/TXC  CRYSTAL'3225'  [4P-SMD-3.2X2.5]

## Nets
2G_ANT: C82.1 R1.1 U14.19(ANT)
2G_XTAL1: U7.B4(RF:XTAL1) X3.1
2G_XTAL2: U7.B5(RF:XTAL2) X3.3
5V_OUT: C1.1 C28.1 C90.1 C108.1 C154.1 C155.1 C156.+ J1.3 J11.3 L24.2 U11.28(5V) U19.3(IN)
/M_SCL: Q4.2(S) R99.2 U7.B11(BB:SCL28)
/M_SDA: Q3.2(S) R98.2 U7.C7(BB:SDA28)
/SPI_MISO: U6.7(NO3) U18.8(A7)
/SPI_MOSI: U6.15(NO1) U18.7(A6)
/SPI_SCL: R108.1 U6.3(NO2) U18.9(A8)
/SPI_SS: U7.B13(BB:CMPDN) U18.6(A5)
ACCDET: R14.2 U7.K5(ABB:ACCDET)
AD0/D14: R88.2 U11.19(PC0/AD0/D14)
AD1/D15: R89.2 U11.20(PC1/AD1/D15)
AD2/D16: R90.2 U11.21(PC2/AD2/D16)
ADC3: U11.22(PC3/AD3/D17)
ANTSEL_0: C143.1 U1.K8(ANTSEL_0) U16.1(VCONT1)
ANTSEL_1: C144.1 U1.J8(ANTSEL_1) U16.3(VCONT2)
APC_VBAIS: R57.2 U7.N7(RF:APC)
AUDIO_GND: D4.2 J16.2 R25.2
AVDD_SMPS: C12.1 C151.1 L2.2 U1.A2(AVDD43_REF) U1.A4(AVDD43_SMPS)
BANDSW: R60.2 U7.D5(RF:BPI_BUS0)
BAT_CHARGE: R94.1 SW3.CH2A
BATON: R84.1 U7.H5(ABB:BATON)
BATTERY: C109.1 J2.+ SW3.CH1A
BPI_BUS2: R67.2 R85.2 U7.A12(RF:BPI_BUS2)
BT_ANT: C110.1 C111.1 C145.2 L14.2
BT_LNA: C114.1 L12.1 U7.A6(RF:BT_LNA)
BUCK_VBAT: C78.2 C79.1 L13.1 R34.2 SW3.CH1B SW3.CH2B
CHR_LDO: C48.1 Q1.1(G) R93.2 U7.G5(ABB:CHRLDO)
CLDO: C21.1 C22.1 U1.C1(CLDO) U1.G4(PAD_VDDK) U1.G6(PAD_VDDK) U1.G7(PAD_VDDK)
CMCSD0: U6.4(COM2) U7.A13(BB:CMCSD0)
CMCSD1: U6.16(COM1) U7.E5(BB:CMCSD1)
CMMCLK: U6.8(COM3) U7.B9(BB:CMMCLK)
CMRST/EINT15: U7.B10(BB:CMRST) U18.3(A2)
D8/GPIO48/EINT21: Q12.3(D) R117.1 U11.9(PB0/D8)
DRV: Q1.2(S) U7.J2(ABB:DRV)
EAR_EINT: R40.1 U7.A3(BB:EINT)
EINT_WIFI: R6.1 U1.E2(WI-FI_INT_B) U7.C8(BB:CMCSK)
FB_OUT: C4.1 C88.+ C153.1 D7.- L24.1 R62.1
FM_ANT_P-1: L11.1 R25.1 R104.1 U7.F2(RF:FM_ANT_P)
FREF_26M_WIFI: C20.1 U7.A5(RF:FREF)
GND: C1.2 C2.2 C3.2 C4.2 C5.2 C6.2 C7.2 C8.2 C9.2 C10.2 C11.2 C12.2 C13.1 C14.1 C15.2 C16.1 C17.1 C18.1 C19.1 C21.2 C22.2 C23.2 C26.2 C27.2 C28.2 C29.2 C30.- C32.2 C33.- C34.2 C35.2 C36.2 C37.2 C38.2 C39.2 C40.2 C41.2 C42.2 C44.2 C45.2 C46.2 C47.2 C48.2 C49.- C50.- C53.2 C54.2 C56.2 C57.2 C60.2 C61.2 C62.2 C63.2 C64.2 C65.2 C66.2 C68.2 C69.2 C70.2 C71.2 C72.2 C73.2 C74.2 C75.2 C76.2 C77.2 C79.2 C80.2 C81.2 C82.2 C83.2 C84.2 C87.2 C88.- C89.2 C90.2 C91.2 C92.2 C93.2 C94.2 C95.2 C96.2 C97.2 C98.2 C99.2 C100.2 C101.2 C102.2 C103.2 C104.2 C106.2 C107.- C108.2 C109.2 C110.2 C112.2 C113.2 C114.2 C115.2 C116.2 C117.2 C119.2 C120.2 C122.2 C124.2 C125.2 C126.1 C127.1 C128.1 C129.2 C130.2 C131.2 C132.2 C133.2 C134.2 C135.2 C136.2 C139.2 C140.2 C143.2 C144.2 C148.- C151.2 C152.1 C153.2 C154.2 C155.2 C156.- C157.1 C158.2 D2.1(+) D3.3 D4.3 D6.3 GPS.GND1 GPS.GND2 GPS.GND3 GSM.GND1 GSM.GND2 GSM.GND3 J1.4 J1.SS1 J1.SS2 J2.3 J2.4 J2.- J4.6(VSS) J4.C5(SIM_GND) J4.P1(PAD1) J4.P2(PAD2) J4.P3(PAD3) J4.P4(PAD4) J4.P5(PAD5) J4.SB(SWITCH-B) J7.5(GND) J7.S1(GND) J7.S2(GND) J7.S3(GND) J7.S4(GND) J7.S5(GND) J7.S6(GND) J11.4 J11.SS1 J11.SS2 JTAG.2 JTAG.3 L11.2 L15.1 L18.2 PWR.- Q2.2(S) R3.2 R5.2 R6.2 R15.2 R16.2 R19.1 R24.1 R29.1 R35.2 R45.2 R56.2 R58.2 R59.2 R75.1 R84.2 R85.1 R86.2 R91.1 R96.2 R97.2 R104.2 R109.1 R110.1 RESET.2 RESET.S1 RESET.S2 RX.- SW1.SS1 SW1.SS2 SW1.SS3 SW1.SS4 SW2.B SW2.SS1 SW2.SS2 SW2.SS3 SW2.SS4 TX.- U1.A10(AVSS33_PA) U1.B1(GND_REF) U1.B3(AGND43_SMPS) U1.B8(AVSS16_VCO) U1.B9(AVSS33_PA) U1.C5(GND_PALDO) U1.C6(AVSS16_WF) U1.C9(AVSS33_PA) U1.D4(AVSSRTC) U1.D6(AVSS16_WF) U1.D7(AVSS16_WF) U1.D9(AVSS16_WF) U1.E1(FSOURCE) U1.F4(CGND) U1.F6(CGND) U1.F7(CGND) U1.J9(XTEST) U1.K1(CGND) U2.8(AVSS43_MISC) U2.14(AVSS43_DCV) U2.29(GND) U2.46(XTEST) U2.PAD(HEAT) U3.4(GND) U3.PAD U4.2(VSS) U6.6(GND) U6.PAD U7.A2(RF:AVSS_2GHF) U7.A8(RF:AVSS_2GHF) U7.B6(RF:AVSS_2GHF) U7.C5(RF:AVSS_2GHF) U7.D2(RF:AVSS_2GHF) U7.D3(RF:AVSS_2GHF) U7.D4(RF:EXT_CLK_SEL) U7.E2(ABB:AVSS44_ALDO) U7.F4(BB:TESTMODE) U7.F5(ABB:GND) U7.F6(ABB:GND) U7.F7(ABB:GND) U7.G2(RF:AVSS_FM) U7.G6(ABB:GND) U7.G7(ABB:GND) U7.H6(ABB:GND) U7.H7(ABB:GND) U7.H8(ABB:GND) U7.J5(ABB:AVSS44_PMU) U7.J6(ABB:AVSS28_ABB) U7.J7(ABB:GND) U7.J8(ABB:GND) U7.K1(ABB:AVSS44_PMU) U7.K6(ABB:GND) U7.L1(ABB:AVSS44_BOOST) U7.L2(ABB:AVSS44_BOOST) U7.M3(ABB:AVSS_SPK) U7.M11(ABB:GND) U7.N8(ABB:RTC_XOSC32_ENB) U7.N9(ABB:AVSS44_DLDO) U7.P2(ABB:AVSS_SPK) U9.2(GND) U9.3(GND) U9.5(GND) U10.1 U10.2 U10.3 U10.4 U10.5 U10.6 U10.7 U10.8 U10.9 U10.10 U11.15(GND) U11.26(GND) U11.27(GND) U11.35(GND) U12.4(GND) U13.1(GND) U13.2(GND) U14.1(GND) U14.2(GND) U14.5(GND) U14.6(GND) U14.8(GND) U14.9(GND) U14.10(GND) U14.11(GND) U14.12(GND) U14.13(GND) U14.18(GND) U14.20(GND) U14.21(GND) U14.22(GND) U14.23(GND) U14.24(GND) U14.25(GND) U14.28(GND) U14.32(GND) U14.33(GND) U14.34(GND) U14.35(GND) U14.36(GND) U15.4(GND) U15.6(GND) U15.8(GND) U16.5(GND) U16.PAD(GND) U18.11(GND) U19.1(GND) U20.4(GND) U20.7(FSEL) WI-FI/BT.GND1 WI-FI/BT.GND2 WI-FI/BT.GND3 X2.1 X2.2 X3.2 X3.4
GNSS_CORE_1V1: C37.1 C41.1 C42.1 U2.6(DVDD11_CORE1) U2.13(AVDD11_CLDO) U2.24(DVDD11_CORE2) U2.43(DVDD11_CORE3)
GNSS_DCV: L3.1 U2.15(DCV)
GNSS_DCV_1V8: C34.1 C44.1 L3.2 R80.1 U2.1(AVDD18_RXFE) U2.4(AVDD18_CM) U2.12(AVDD28_CLDO) U2.17(DCV_FB)
GNSS_EN: U4.3(CE) U7.D8(BB:KCOL0)
GNSS_FRAME_SYNC: R26.1 R65.1 U7.B12(BB:KCOL1)
GNSS_HRST: R52.1 U7.H12(ABB:SIM2_SCLK)
GNSS_REF: C38.1 U2.7(VREF)
GNSS_TXIND: U2.25(TX1/TXIND/RTS0/MM_I2CD/CXO_CS/GIO1) U7.E6(BB:KCOL2)
GNSS_UART_RX: U2.35(RX0/MM_I2CC/H_SPI_SI) U7.E13(BB:KROW4)
GNSS_UART_TX: R63.1 U2.37(TX0/MM_I2CD/H_SPI_SO) U7.D10(BB:KCOL4)
GNSS_VGNSS_MAIN: C31.2 C35.1 C39.1 C46.1 U2.9(AVDD43_VBAT) U2.16(AVDD43_DCV) U4.5(VOUT)
GNSS_VRTC_1V1: C31.1 C99.1 U2.18(AVDD11_RTC)
GNSS_VRTC_4V3: C29.1 D1.- R7.1 U2.19(AVDD43_RTC)
GNSS_VTCXO_SW: C26.1 C80.1 C119.1 C120.1 L20.2 R41.2 U2.10(AVDD_TCXO_SW) U13.4(VCC) X2.4
GNSS_VTLDO: C36.1 C40.1 R31.1 U2.11(AVDD28_TLDO) U2.30(DVDD28_IO1) U2.42(DVDD28_IO2)
GPIO0/ADC0/U3RX: C103.1 R59.1 R88.1 U7.F8(BB:GPIO_0) U17.4
GPIO1/ADC1/U3TX: C102.1 R58.1 R89.1 U7.E12(BB:GPIO_1) U17.5
GPIO2/ADC2/PWM0: C89.1 R45.1 R90.1 U7.D11(BB:GPIO_2) U17.2
GPIO13/EINT11/PWM0: R64.1 U7.D12(BB:KCOL3) U18.4(A3)
GPIO19/PWM1: R66.1 U7.C11(BB:KROW2) U18.5(A4)
GPIO40/SIM2_SIO: Q10.2(S) R112.2 U7.J12(ABB:SIM2_SIO)
GPIO_3/PWM1: U7.D13(BB:GPIO_3) U18.1(A1)
GPS_RFIN: C67.2 L18.1 U2.48(RF_IN)
GPS_RTC_32K: U2.21(XIN) U7.J11(ABB:SIM2_SRST)
ISENSE: Q14.3(C) R94.2 U7.H2(ABB:ISENSE) U8.1(C) U8.2(C) U8.5(C) U8.6(C)
JTAG_2V8: JTAG.1 R38.2
JTCK: JTAG.9 R65.2
JTDI: JTAG.7 R63.2
JTDO: JTAG.8 R66.2
JTMS: JTAG.10 R64.2
JTRST_B: JTAG.6 R39.2
JTRTCK: JTAG.4 R68.1
LPTE_MUX: Q13.2(S) R118.2 U7.J10(BB:LPTE)
LSA0_LCM: R24.2 R37.2 U7.J9(BB:LSA0)
LSCE_B/EINT20: Q11.2(S) R114.2 U7.G9(BB:LSCE_B)
LSCK_LCM: R97.1 U7.L10(BB:LSCK)
LSDA_LCM/EINT21: Q12.2(S) R115.2 U7.L11(BB:LSDA)
LSRSTB: R96.1 U7.H9(BB:LSRSTB)
M_SCL: Q4.3(D) R23.2 R73.1 U11.18(SCL) U11.24(PC5/AD5/D19/SCL)
M_SDA: Q3.3(D) R22.2 R71.1 U11.17(SDA) U11.23(PC4/AD4/D18/SDA)
MC2_CLK: J4.5(SD_CLK) U6.1(NC1)
MC2_CMD: J4.3(CMD) U6.5(NC2)
MC2_DA0: J4.7(DAT0) U6.9(NC3)
MCINS: J4.SA(SWITCH-A) U7.D7(BB:KROW0)
MIC1_N: C55.1 U7.N5(ABB:AU_VIN1_N)
MIC1_P: C58.1 U7.P5(ABB:AU_VIN1_P)
MICBIAS0: R12.2 U7.L4(ABB:AU_MICBIAS0)
MP3_OUTL: L9.1 U7.P1(ABB:AU_HPL)
MP3_OUTR: L10.1 U7.N1(ABB:AU_HPR)
N$1: R87.1 U1.F8(ANTSEL_3)
N$2: C27.1 C85.1 R79.1
N$3: R92.1 U1.G9(ANTSEL_2)
N$4: R69.2 U18.10(OE)
N$5: J4.1(DAT2) R74.2
N$6: C24.1 U9.1(INPUT)
N$7: C6.1 U1.A1(REF)
N$8: C20.2 U1.A7(OSC_IN)
N$9: C15.1 R4.2 U1.A6(AVDD33_XO)
N$10: C85.2 GPS.D L20.1
N$11: J1.1 R28.1
N$12: L6.2 U1.A3(LXBK)
N$13: L5.2 U13.3(RFIN)
N$14: C25.1 U9.4(OUTPUT)
N$15: J11.1 R23.1
N$16: C43.1 U2.5(OSC)
N$17: C148.+ R7.2
N$18: R41.1 U13.5(!SHDN)
N$20: R19.2 SW1.B
N$22: D7.+ L8.2 U20.5(LX)
N$23: J1.2 R27.1
N$24: C51.1 L9.2
N$25: C52.1 L10.2
N$26: C51.2 R10.1
N$27: C52.2 R11.1
N$28: C55.2 C57.1 C59.2 C60.1 R12.1 R13.2
N$29: C96.1 U7.N10(ABB:VIBR)
N$30: Q6.3(D) RX.+
N$31: R47.1 U7.H10(ABB:RESETB)
N$32: D15.- U11.30(RESET)
N$33: C84.1 R21.1 WI-FI/BT.D
N$34: R33.2 U12.6(EN/SYNC)
N$35: R30.2 U20.1(COMP)
N$36: C157.2 R30.1
N$38: R62.2 R91.2 U20.2(FB)
N$39: Q6.2(S) R76.1
N$40: J11.2 R22.1
N$41: J4.2(CD/DAT3) R2.2
N$42: C115.1 C137.1 R21.2
N$43: Q7.2(S) R77.1
N$44: R48.1 U12.5(BS)
N$45: C105.2 R48.2
N$46: R50.1 U12.8(FB)
N$47: C77.1 U12.7(VCC)
N$48: C78.1 R51.2
N$49: C104.1 U7.D1(ABB:VRF)
N$50: C105.1 L13.2 U12.3(SW)
N$51: C100.1 U12.1(SS)
N$52: R34.1 R35.1 R50.2 R51.1
N$55: J16.1 L21.2
N$56: PWR.+ R78.1
N$57: R36.1 RST.+
N$58: R52.2 U2.47(HRST_B)
N$59: C158.1 U20.8(SS)
N$60: J4.8(DAT1) R72.2
N$61: R26.2 U2.33(FRAME_SYNNC/DBG_RX/GIO8)
N$62: C113.1 L4.1 L12.2 L14.1
N$63: C112.1 L4.2
N$64: C43.2 X2.3
N$65: C25.2 L5.1
N$66: C111.2 L15.2
N$67: C118.1 U13.6(RFOUT)
N$68: C67.1 C68.1 C118.2
N$69: R31.2 U2.32(RX2/SPI_SI/JDI/DBG_RX/BSI_CK/GIO2)
N$70: R80.2 U2.40(BSI_CS/MM_I2CD/DUTY_CYCLE/PPS/GIO7)
N$71: J16.6 R40.2 R53.1
N$72: C124.1 GSM.D R54.1
N$73: C83.1 C125.1 R1.2 R54.2
N$74: C130.1 R55.1 U14.31(TX_EN)
N$75: C131.1 R56.1 R57.1 U14.30(VRAMP)
N$76: C132.1 L17.1 U14.16(RX_LB)
N$77: C133.1 L19.1 U14.15(RX_HB)
N$78: Q1.3(D) Q14.1(B) U8.3(B)
N$80: L1.1 U14.4(RFIN_LB)
N$81: L16.1 U14.3(RFIN_HB)
N$82: C136.1 U14.7(VBAT2)
N$83: C129.1 R60.1 U14.29(SW1)
N$84: C93.1 C107.+ R8.2
N$85: C138.2 U15.1(UNBALANCED_PORT)
N$86: Q7.3(D) TX.+
N$88: C138.1 U16.6(OUTPUT1)
N$89: C145.1 U16.4(OUTPUT2)
N$90: C137.2 U16.2(INPUT)
N$91: L.+ R49.1
N$94: L.- Q2.3(D)
N$95: R20.2 SW1.A
N$104: R105.2 SW2.A SW2.COM
N$105: C24.2 C117.1 R79.2
N$106: J16.4 L22.2
N$107: J16.3 J16.7 L23.2
N$108: Q6.1(G) R106.1
N$109: Q7.1(G) R107.1
N$110: Q2.1(G) R29.2 R108.2
N$111: R109.2 U2.31(SCK1/SPI_SCK/GIO4)
N$112: R110.2 U2.41(SCS1#/SPI_SCS#/BSI_DATA/SYNC_PULSE/GIO5)
PALDO_3V3: C18.2 C139.1 C140.1 C152.2 R4.1 U1.A5(PALDO) U1.A9(AVDD33_TX) U1.E5(PALDO_FB) U15.2(NC/DC_FEED) ; supply symbol labelled POWER_CIRCLE
PB1/D9/PWM1: U11.10(PB1/D9/PWM) U18.16(B4)
PD0/RX: Q9.3(D) R28.2 R111.1 U11.1(PD0/D0/RX)
PD1/TX: Q8.3(D) R27.2 R83.1 U11.2(PD1/D1/TX)
PD2/INT0: Q11.3(D) R116.1 U11.3(PD2/D2/INT0)
PD3/INT1/PWM0: U11.4(PD3/D3/INT1/PWM) U18.17(B3)
PD4: Q10.3(D) R113.1 U11.5(PD4/D4)
PD5/PWM: U11.6(PD5/D5/PWM) U18.20(B1)
PD6/PWM: U11.7(PD6/D6/PWM) U18.18(B2)
PD7: Q13.3(D) R119.1 U11.8(PD7/D7)
PWRKEY: R105.1 U7.G4(ABB:PWRKEY)
RESET: C81.1 D15.+ JTAG.5 R47.2 R81.1 RESET.1 RST.-
RXHB_P: L19.2 U7.B1(RF:RXHB)
RXLB_P: L17.2 U7.A1(RF:RXLB)
SIM1_SCLK: C62.1 J4.C3(SIM_CLK) U7.K7(ABB:SIM1_SCLK)
SIM1_SIO: C64.1 J4.C7(I/O) U7.L9(ABB:SIM1_SIO)
SIM1_SRST: C61.1 J4.C2(RST) U7.K8(ABB:SIM1_SRST)
SMPSLDO_1V6: C11.1 C13.2 C16.2 C17.2 C19.2 L6.1 U1.A8(AVDD16_SX) U1.C2(AVDD16_CLDO) U1.C3(OUT_FB) U1.D10(AVDD16_TRX) U1.E10(AVDD16_LF)
SPI_MISO: U11.13(PB4/D12/MISO) U11.38(MISO) U18.13(B7)
SPI_MOSI: U11.12(PB3/D11/MOSI/PWM) U11.34(MOSI) U18.14(B6)
SPI_SCL: U11.14(PB5/D13/SCK) U11.37(SCK) U18.12(B8)
SPI_SS: U11.11(PB2/D10/SS/PWM) U18.15(B5)
SQI_CE: U3.1(CS#) U7.G13(BB:SFSCS0)
SQI_SCK: U3.6(SCLK) U7.G8(BB:SFSCK)
SQI_SI: U3.5(SI/SIO0) U7.F9(BB:SFSOUT)
SQI_SIO2: U3.3(WP#/SIO2) U7.F12(BB:SFSWP)
SQI_SIO3: U3.7(RESET#SIO3) U7.F10(BB:SFSHOLD)
SQI_SO: U3.2(SO/SIO1) U7.G12(BB:SFSIN)
SW_SPI/SDIO: SW1.COM U6.2(INA) U6.10(INB)
TR_N: C141.1 L7.1 U15.7(BALANCED_PORT)
TR_P: C141.2 R61.1 U15.5(BALANCED_PORT)
TRX_IO_N: C142.1 L7.2 U1.C10(TRX_IO_N)
TRX_IO_P: C142.2 R61.2 U1.B10(TRX_IO_P)
TX_EN: R55.2 R75.2 U7.A9(RF:BPI_BUS1)
TXO_HB: C134.1 L16.2 U7.C2(RF:TX_HB)
TXO_LB: C135.1 L1.2 U7.B2(RF:TX_LB)
UART1_RX: Q9.2(S) R82.2 R106.2 U7.E9(BB:URXD1)
UART1_TX: Q8.2(S) R46.2 R107.2 U7.E8(BB:UTXD1)
USB_5V: C49.+ C74.1 C98.1 C106.1 C116.1 J7.1(VCC) Q14.2(E) R33.1 R70.1 R93.1 U8.4(E) U12.2(IN) VCHG_5V1.T
USB_N: DP.T J7.2(DM) R17.1
USB_P: DN.T J7.3(DP) R18.1
USBD_N: D6.1 R17.2 U7.N11(BB:USB11_DM)
USBD_P: D6.2 R18.2 U7.P11(BB:USB11_DP)
VA: C94.1 U7.P3(ABB:VA)
VBAT: C3.1 C8.1 C30.+ C33.+ C45.1 C50.+ C72.1 C73.1 C101.1 C126.2 C127.2 C128.2 D2.2(-) L2.1 L8.1 R78.2 SW3.COM1 SW3.COM2 U4.1(VIN) U7.E1(ABB:VBAT_VA) U7.H1(ABB:BATSNS) U7.L3(ABB:AVDD_SPK) U7.M10(ABB:VBAT_DIGITAL) U14.26(VBAT1) U20.3(EN) U20.6(VDD) VBAT_TP.T
VCDT: R70.2 R86.1 U7.J4(ABB:VCDT)
VCORE: C69.1 U7.A11(ABB:VDDK) U7.P9(ABB:VCORE)
VIO18_LDO: C70.1 Q11.1(G) Q12.1(G) Q13.1(G) R37.1 R114.1 R115.1 R118.1 U7.N13(ABB:VIO18) U7.P13(ABB:VIO18)
VIO28_LDO: C5.1 C14.2 C23.1 C63.1 C71.1 C122.1 Q3.1(G) Q4.1(G) Q8.1(G) Q9.1(G) Q10.1(G) R36.2 R38.1 R46.1 R49.2 R53.2 R67.1 R69.1 R76.2 R77.2 R81.2 R82.1 R87.2 R92.2 R98.1 R99.1 R112.1 U1.D3(AVDDRTC) U1.H1(DVDDIO3) U1.J7(DVDDIO2) U1.K7(DVDDIO1) U1.K10(DVDDIO0) U7.B7(RF:AVDD15_BTRF) U7.B8(ABB:VIO28) U17.3 U17.6 U18.2(VCCA) VIO_28.T
VIO33_LDO: C2.1 C7.1 C32.1 C87.1 R20.1 R71.2 R73.2 R83.2 R111.2 R113.2 R116.2 R117.2 R119.2 U6.14(VCC) U11.29(3V3) U11.31(ADC7) U18.19(VCCB) U19.2(OUT) U19.4(OUT)
VMC: C66.1 C95.1 J4.4(VDD) R2.1 R72.1 R74.1 U7.K9(ABB:VMC)
VREF: C92.1 U7.G1(ABB:VREF)
VRTC: D1.+ R8.1 U7.P8(ABB:VRTC)
VSF: C47.1 C91.1 U3.8(VCC) U7.F11(ABB:VSF)
VSIM1: C65.1 C97.1 J4.C1(VCC) J4.C6(VPP) U7.L7(ABB:VSIM1)
VSIM2: C9.1 U7.H13(ABB:VSIM2)
VUSB: C10.1 U7.P12(ABB:VUSB)
WIFI_BT_PRI: R5.1 R68.2 U1.H7(BT_PRI) U7.C12(BB:KROW1)
WIFI_EN: R3.1 U1.B5(PAD_EN) U7.C3(BB:GPIO_10)
WIFI_MC1CLK: U1.J2(OE_N) U7.K12(BB:MCCK)
WIFI_MC1CMD: U1.J1(A0) U7.L13(BB:MCCM0)
WIFI_MC1DA0: U1.H3(D0) U7.K13(BB:MCDA0)
WIFI_MC1DA1: U1.J3(D1) U7.M12(BB:MCDA1)
WIFI_MC1DA2: U1.H2(D2) U7.L12(BB:MCDA2)
WIFI_MC1DA3: U1.K2(D3) U7.N12(BB:MCDA3)
WIFI_OSC_EN: U1.F9(OSC_EN) U7.B3(BB:SRCLKENAI)
WIFI_RST_N: U1.K9(SYSRST_B) U7.C4(BB:GPIO_11)
WIFI_RTC: R32.2 R39.1 U7.E7(BB:KROW3)
WIFI_XIN: R32.1 U1.D1(X32K_IN)
XIN: C75.1 U7.M7(ABB:XIN) X1.1
XMIC: C56.1 C58.2 C59.1 D3.2 L21.1 R13.1 R14.1
XMP3_L: C54.1 D3.1 L22.1 R10.2 R16.1
XMP3_R: C53.1 D4.1 L23.1 R11.2 R15.1
XOUT: C76.1 U7.M6(ABB:XOUT) X1.2
Unconnected: J7.4(ID) J16.5 J16.8 U1.D2(X32K_OUT) U1.E3(D7) U1.E6(TRX_IP) U1.E7(TRX_IN) U1.E8(TRX_QP) U1.E9(TRX_QN) U1.F2(WE_N) U1.F3(CS_N) U1.F10(PAD_ICAL_EXTR) U1.G1(D4) U1.G2(D5) U1.G3(D6) U1.G10(GPIO_0) U1.H4(D10) U1.H5(D11) U1.H6(D12) U1.H8(EXT_INT_B) U1.H9(GPIO_1) U1.H10(UART_DBG_RX) U1.J4(D9) U1.J5(D14) U1.J6(D15) U1.J10(UART_DBG_TX) U1.K4(D8) U1.K6(D13) U2.2(T1P) U2.3(T1N) U2.20(XOUT) U2.22(FORCE_ON) U2.23(32K_OUT/DR_IN) U2.26(BSI_CK/MM_I2CC/ECLK/GIO6) U2.27(RX1/H_SPI_SCK/CTS0/MM_I2CC/CXO_TSENS/GIO0) U2.28(TX2/SPI_SO/DBG_TX/GIO3) U2.34(CXO_CS/GIO10) U2.36(EINT2/DBG_RX/PPS/GPIO14) U2.38(H_SPI_SCS#/CXO_TSENS/SYNC_PULSE/GIO11) U2.39(PPS/DBG_TX/GIO9) U2.44(EINT0/MM_I2CC/SBI_CS/GIO12) U2.45(EINT1/MM_I2CD/PPS/BSI_DATA/GIO13) U4.4(NC) U6.11(NO4) U6.12(COM4) U6.13(NC4) U7.F3(ABB:VCAMA) U7.J3(ABB:KPLED) U7.K2(ABB:ISINK) U7.L6(BB:AUXIN4) U7.M2(ABB:SPK_OUTN) U7.N2(ABB:SPK_OUTP) U7.N3(ABB:AU_HSP) U7.N4(ABB:AU_HSN) U7.N6(ABB:AU_VIN0_N) U7.P6(ABB:AU_VIN0_P) U11.16(AREF) U11.25(VIN) U11.32(ADC6) U11.33(VCC) U11.36(RST) U14.14(NC) U14.17(NC) U14.27(NC) U15.3(NC) U17.1

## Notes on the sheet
- SYS CONFIG
- direct to GND plane of charge pump
- RESET KEY
- FOR ESD
- YiLong.Qin | Bruce Qin
- v0.9
- SD Card/ SPI
- JTAG
- KCOL3
- KCOL1
- IO INTERFACE
  CONFIG
- KROW2
- KROW1 | KCOL4
- KROW3
- HW bootup
- BAT DET | disabled test mode
- Serial Flash
- WIFI
- 0:VSF 1V8
- 1:VSF 3V0 | 500mA
- JTAG MODE
- USB UART
- USB MASS Storage
- JTAG MODE   R67     NC/R85
  NORMAL      NC/R67  R85
- YiLong.Qin | Bruce Qin
- v0.9
- POWER
- Reserved
- BATTERY
- LOW   T-card  (defualt)
  High   SPI
- U10 & Q2 compatibility | differential line
- DCDC 5V TO 4.2V
- SD | SPI
- BAT
- DCDC
- YiLong.Qin | Bruce Qin
- v0.9
- EXTEND INTERFACE
- GPIO Interface
- 2.8V | 1.8V
- D4 | D7
- SPI Interface
- UART_RX | D8
- UART_TX | D2
- IIC_SCL
- 500mA
- IIC_SDA
- YiLong.Qin | Bruce Qin
- v0.9
- must close to 2502
  the max trace is 80mil
- GSM/GPRS
- C63 close to MT2502 B7
- must close to PA
  the max trace is 50mil
- YiLong.Qin | Bruce Qin
- v0.9
- GPS
- Option: 3V3 supply for active ANT
- 200mA
- close to GPS AVDD43_DCV [PIN16] | close to GPS AVDD11_CLDO [PIN13]
- 16.368MHZ TCXO : R109 = NC , R110 = NC
- 26MHZ TCXO : R109 = 10K , R110 = NC
- 26MHZ XTAL : R109 = 10K , R110 = 10K
- YiLong.Qin | Bruce Qin | YiLong.Qin | Bruce Qin
- v0.9 | v0.9
- WIFI/BT
- close to MT2502
- optional for better BT
- close to AVDD16_SX [A8] | close to AVDD33_TX [A9] | close to AVDD16_TRX [D10] | close to AVDD16_LF [E10] | close to AVDDRTC [D3] | close to AVDD16_CLDO [C2]
- YiLong.Qin | Bruce Qin | YiLong.Qin | Bruce Qin
- v0.9 | v0.9
- SERIAL FLASH & SD CARD
- Serial Flash
- SD Interface
- SIM
- TF card OUT --SWITCH OPEN
  TF card IN  --SWITCH CONTACT
- YiLong.Qin | Bruce Qin
- v0.9
- AUDIO INTERFACE
- AUDIO
- YiLong.Qin | Bruce Qin
- v0.9
- USB&SIM INTERFACE
- USB | UART Interface
- IIC Interface
- YiLong.Qin | Bruce Qin
- v0.9

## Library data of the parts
C1-C29 C31 C32 C34-C48 C51-C85 C87 C89-C106 C108-C120 C122 C124-C145 C151-C155 C157 C158 = Discrete:C*: Ceramic Capacitors
C30 C33 C49 C50 C88 C156 = Discrete:CAP*: Electrolytic Capacitors,Tantalum Capacitors and Super Capacitors
C107 C148 = template:C-ELECTRIC-DOUBLE-LAYER-CAPACITOR: Electric Double Layer Capacitor
D1 D7 D15 = Discrete:D*
D2 = Discrete:D-VOL
D3 D4 D6 = Discrete:D-ESD-3P
DN DP VBAT_TP VCHG_5V1 VIO_28 = Discrete:PAD-TEST-POINT; PARTNO: DNP
GPS GSM WI-FI/BT = Connector :ANTENNA-U-FL
J1 J11 = Connector :TWIG-4P-2.0-SMD-FEMALE-REINFORCE
J2 = Connector :JACK-JST-2P-SMD-PW
J4 = template:HOLDER-SD/SIM-CONNECTER: T-FLASH+SIM
J7 = Connector :USB-MINIUSB-5P
J16 = Connector :AUDIO-8P-SMD
JTAG = template:HEADER-2X5P-2.0
L PWR RST RX TX = Discrete:LED*
L1-L24 = Discrete:L*
P1-P12 = Discrete:PAD-MARK; PARTNO: DNP
Q1-Q4 Q8-Q13 = Discrete:MOSFET-N: IRLL014: http://www.vishay.com/docs/91319/sihll014.pdf
Q6 Q7 = Discrete:MOSFET-P
Q14 = Discrete:TRANSISTOR-PNP*: PNP audion
R1-R8 R10-R41 R45-R94 R96-R99 R104-R119 = Discrete:R*
RESET = Discrete:BUTTON-4P-REINFORCE: TS-1188E http://www.best-dz.com/?thread-374-2.html
SW1 SW2 = Discrete:SWITCH-3P-SMD
SW3 = Discrete:SWITCH-2CH-6P
U1 = template:MT5931: MT5931 is a Wi-Fi device which includes 802.11 b/g/n \ PA \ LNA \ TR-Swithch
U2 = template:MT3332: MT3332 is a high-performance single-chip multi-GNSS solution which includes on-chip CMOS RF and digital baseband.
U3 = template:MX25U12835F: 1.8V 128M-BIT[X1/X2/X4]CMOS MXSMIO(SERIAL MULTI I/O) FLASH MEMORY
U4 = IC:XC6228: 300mA High Speed LDO Regulator with ON/OFF Switch
U6 = template:BCT4699: 0.5 OU .3.3V Quad-SPDT Analog Switch
U7 = template:MT2502A: SOC processor Technical Brief
U8 = template :STT818B: High Gain Low Voltage PNP Power Transistor
U9 = template :FILTER-FOR_GPS1500
U10 = template:SHIELDING-COVER
U11 = moudle:ARDUINO-38P
U12 = template :MP1496DJ: High-Efficiency,2A，16V,500kHz Synchronous,Step-Down Converter http://html.alldatasheetcn.com/html-pdf/551584/MPS/MP1496DJ/55/1/MP1496DJ.html
U13 = template :MAX2659: GPS/GNSS Low-Noise Amplifier
U14 = template :RF1798: Quad-Band GSM850/GSM900/DCS1800/PCS1900 TX Module
U15 = template :FILTER-FB2012: FB2012 Series Multilayer Chip Band Pass Filter+Balun
U16 = template :UPG2176T5N: 50 OU TEMRMINATON TYPE HIGH POWER SPDT SWITCH FOR WIMAX
U17 = template:BAV70S: High-speed double diode array
U18 = template:TXS0108E: 8-BIT BIDIRECTIONAL VOLTAGE-LEVEL TRANSLATOR FOR OPEN-DRAIN AND PUSH-PULL APPLICATIONS
U19 = IC:LD1117: Low Drop Fixed And Adjustable Positive Voltage Regulators http://www.datasheetcatalog.org/datasheet/SGSThomsonMicroelectronics/mXuqtqv.pdf
U20 = IC:ISL97516
X1 = Discrete:CRYSTAL*: CRYSTAL
X2 X3 = template :CRYSTAL

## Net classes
0 default: width 0.076 mm, drill 0.102 mm, clearance 0.076 mm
